(* Logix 5000 Rung export; software revision 16.04 *)

MODULES
   Local : vendor None type None code None
   DNPNET : vendor None type None code None
END_MODULES

TYPE DNPNET_A32in_ClassDeadband_Override :   // List entry for Analog32 Input Class and Deadband Override
STRUCT
   Point_Number : INT;   // Point number to assign class and deadband to.
   Class : INT;   // Class value (1-3)
   Deadband : DINT;   // Deadband for given point number
END_STRUCT
END_TYPE

TYPE DNPNET_CROBmsg_Handler :   // Handles the processing of CROB Messages from Remote Client
STRUCT
   OneShot : BOOL;
   CountPerBlock : INT;   // Number of CROB messages from the Remote Client in in the last 9910 block of multiple blocks.
   CCC : DINT;   // Continuous Crob message Count that may be reset by the User. Otherwise it will cycle from 0 to the DINT type upper limit
   CCBC : DINT;   // Continuous Crob Message Block Count that may be reset by the User. Otherwise it will cycle from 0 to the DINT type upper limit
END_STRUCT
END_TYPE

TYPE DNPNET_Server_List :   // List entry to define an IED unit and its specific communication parameters for a DNP Client port
STRUCT
   Address : INT;
   Data_Link_Confirm_Mode : INT;
   Data_Link_Confirm_Timeout : INT;
   Data_Link_Confirm_Retries : INT;
   Application_Layer_Response_Timeout : INT;
   Server_Mode : INT;   // Bit 0: Enable; Bit 1: Unsol. Msg; Bit 2: Delay Meas; Bit 3: Auto Time Sync; Bit 4: Time Sync Var (0=Var3, 1=Var1)
   IP_Address : DNPNET_WhiteList_IP_address;
   Port : DINT;
   IP_Type : INT;
   Connection_Retry_Interval : INT;
END_STRUCT
END_TYPE

TYPE DNPNETSTATUS :   // This structure encapsulates all the status and scratch variables used by the MVI56E-DNPNET module.
STRUCT
   GenStat : DNPNET_Server_Status;   // General status information
   ErrorList : INT[60];   // List of last 60 DNPNET module errors
   IINServerBits : INT[40];   // IIN Bits received from Servers
   ServerCommErrors : DNPNET_Server_Comm_Error_Element[40];   // Server communication errors list
   CommandErrors : INT[300];   // Command errors list
   Network : DNPNET_Network;
END_STRUCT
END_TYPE

TYPE DNPNET_Command_Error_Request :   // this goes into a 9950 block to request command errors
STRUCT
   Request : BOOL;   // send a 9950 command error request block
   Number_Of_Commands : INT;   // Number of commands to report (1 - 200)
   Start_Index : INT;   // Index in the command list to start
END_STRUCT
END_TYPE

TYPE DNPNETCONTROL :
STRUCT
   Events : DNPNET_EventsHandler;   // Handling the transfer of events from the Events Message Buffer in the Client to the PLC
   EventMessages : DNPNET_EventMessage[15];   // Events Captured by DNP Client are moved to this structure
   CROBmsg_counter : DNPNET_CROBmsg_Handler;   // Number of block 9910 CROB messages from DNP Server
   CROBmsg_data : DNPNET_CROB_Data[40];   // CROB message data copied via block 9910 from DNP Server
   Binary_Event_CalTime : DNPNET_Event_Binary_CalTime;   // For storing block 9958 Binary Input Events with CAL time to be sent by DNP Server
   Analog_Event_CalTime : DNPNET_Event_Analog_CalTime;   // For storing block 9959 Analog Input Events with CAL time to be sent by DNP Server
   Binary_Event_CLXTime : DNPNET_Event_Binary_CLXTime;   // For storing Block 9968 Binary Input Events with CLX Time to be sent by DNP server
   Analog_Event_CLXTime : DNPNET_Event_Analog_CLXTime;   // For storing Block 9969 Binary Input Events with CLX Time to be sent by DNP server
   Get_Module_Time : DNPNET_Module_Time_Get;
   Set_Module_Time : DNPNET_Module_Time_Set;
   CROB_Commands : DNPNET_CROB_Commands;   // 9901 block of CROB Commands
   Aux_Commands : DNPNET_Aux_Command;   // 9904 block for Auxiliary Client commands
   CommandControl : DNPNET_Command_Control;   // 9902 block of commands to enable
   Server_Comm_Errors : DNPNET_Server_Error_Request;   // count and offset of servers to report
   Command_Errors : DNPNET_Command_Error_Request;   // count and offset of commands to report
   ColdBoot : BOOL;   // Cold boot the DNP module via block 9999
   WarmBoot : BOOL;   // Warm boot the DNP module via block 9998
   ChangeDatabaseSize : BOOL;   // Manual bit to change database size
END_STRUCT
END_TYPE

TYPE DNPNET_CROB_Command_Element :   // This is a single CROB command for a CROB command block
STRUCT
   Port_Flag : INT;   // ignored
   Server_Address : INT;   // Address of server to be controlled
   Object : INT;   // Object type 12
   Variation : INT;   // Variation1
   Function : INT;   // Function 3, 5, or 6
   Point_Number_In_Server : INT;   // Point number in the IED to be controlled
   Control_Code : INT;   // Standard DNP control code byte
   Pulse_Count : INT;   // Number of pulses from 0 to 255
   Pulse_On : INT;   // Pulse on time interval
   Pulse_Off : INT;   // Pulse off time interval
END_STRUCT
END_TYPE

TYPE DNPNET_Event_Analog_CalTime :   // Holds binary input events with calendar time block 9959
STRUCT
   Send : BOOL;   // Sends block 9959 Analog_Event messages to DNP Server
   Event_Count : INT;   // Number of events (1 to 20)
   Sequence_Counter : INT;   // Sequence counter for each block transfer, used to synchronize and confirm receipt of the block by the module
   Event : DNPNET_Event_Analog_CalTime_Element[20];   // Analog input events to be transferred to the module
   Event_Count_Rec : INT;   // Number of events (1 - 20) received
   Seq_Count_Rec : INT;   // Sequence counter Received for each block transfer, used to synchronize and confirm receipt of the block by the module
END_STRUCT
END_TYPE

TYPE DNPNET_Event_Binary_CLXTime_Element :   // Block 9968 binary CLXTime event element
STRUCT
   Point_Number : INT;   // Point number in the DNP binary input database
   Class_Override : INT;   // Bits 0 and 1 are used for class override values of 1 to 3
   Value : INT;   // Bit 0 = digital state for point. ALL other bits are ignored
   reserved : INT;
   CLX_Time : LINT;   // 64-bit Time as number of microseconds since Jan 1st, 1970
END_STRUCT
END_TYPE

TYPE DNPNET_DBLin_ClassDeadband_Override :   // List entry for Double Float Input Class and Deadband Override
STRUCT
   Point_Number : INT;   // Point number to assign class and deadband to
   Class : INT;   // Class value (1-3)
   Deadband : REAL;   // Deadband for given point number
END_STRUCT
END_TYPE

TYPE DNPNET_Server_Comm_Error_Element :   // Server communication errors
STRUCT
   Index : INT;   // index in the module's server list
   Server_Address : INT;   // DNP server address for the device
   Bad_CRC : INT;   // number of bad CRCs received from the server
   Buffer_Overflow : INT;   // number of buffer overflow messages received from the server
   Trans_Seq_Num : INT;   // the number of incorrect transport sequence errors
   Confirm_Retry : INT;   // number of data link layer confirm request retries
   Confirm_Fail : INT;   // number of data link layer confirm request failures
   No_App_Resp : INT;   // number of application layer no responses to requests
END_STRUCT
END_TYPE

TYPE DNPNET_WhiteList_IP_address :   // Structure containing the four octets for White List IP addresses
STRUCT
   a : INT;   // a . XXX . XXX . XXX
   b : INT;   // XXX . b . XXX . XXX
   c : INT;   // XXX . XXX . c . XXX
   d : INT;   // XXX . XXX . XXX . d
END_STRUCT
END_TYPE

TYPE DNPNET_Client_Parameters :   // This structure contains configuration parameters for the DNP client
STRUCT
   Internal_ID : INT;   // Client's Identification Number
   Event_Messages_to_PLC : INT;
   Initialize_IED_Input_Database : INT;
   Only_Time_Sync_Servers_If_Synced : INT;
   Use_Binary_Output_status_Data : INT;
   Use_Analog_Output_status_Data : INT;
   Dont_Process_IIN : INT;
   reserved_0 : INT;
END_STRUCT
END_TYPE

TYPE DNPNET_Module_Time_Set :   // Write to Module's System TIme
STRUCT
   Send : BOOL;   // Send block 9971 Time from the PLC to the DNP module
   PLC_Time : DINT[7];   // WallclockTime is copied to this tag before being sent to DNP Module
END_STRUCT
END_TYPE

TYPE DNPNET_Client_Commands :   // List entry for commands to process on the master port
STRUCT
   Port_Flags : INT;   // Bit 2:(0=Disable Cmd, 1=Enable Cmd); Bit 3:(0=Poll, 1=Exception); Bit 4:(0=DNP DB, 1=IED DB). Bits 3/4 apply to BO/AO only.
   Server_Address : INT;   // address of server command is sent to
   Object : INT;   // Object number
   Variation : INT;   // Variation number
   Function : INT;   // Function number
   Point_Number_in_Server : INT;   // starting point for request in server
   Point_Count : INT;   // number of points requested in server
   DNP_DB_Point_Number_in_Client : INT;   // starting point in DNP database for storing response
   IED_DB_Point_Number_in_Client : INT;   // starting point in IED database for storing response
   Poll_Interval : INT;   // how often to send command
END_STRUCT
END_TYPE

TYPE DNPNET_IED_DB_Definitions :   // This structure contains CALCULATED Point Counts/Sizes used by the IED Database. NOT editable by user.
STRUCT
   Binary_Input_Words : INT;   // number of Object 1 words (points * 16)
   Analog16_Inputs : INT;   // number of Object 30 INTs
   Analog32_Inputs : INT;   // number of Object 30 DINTs
   Float_Inputs : INT;   // number of Object 30 REALs
   Counters : INT;   // number of Object 20 DINTs
   Binary_Output_Words : INT;   // number of Object 12 words (points * 16)
   Analog16_Outputs : INT;   // number of Object 41 INTs
   Analog32_Outputs : INT;   // number of Object 41 DINTs
   Float_Outputs : INT;   // number of Object 41 REALs
   Binary_Out_Words_Status_Size : INT;   // number of Object 10 words (points * 16)
   Analog16_Out_Status_Size : INT;   // number of Object 40 INTs
   Analog32_Out_Status_Size : INT;   // number of Object 40 DINTs
   Float_Out_Status_Size : INT;   // number of Object 40 REALs
   reserved_0 : INT;
END_STRUCT
END_TYPE

TYPE DNPNET_IED_Output_Database :
STRUCT
   Binary : INT[100];   // Object 12 binary INTs for Remote Server's database
   Analog16 : INT[100];   // Object 41 analog INTs for Remote Server's database
   Analog32 : DINT[50];   // Object 41 analog DINTs for Remote Server's database
   Float : REAL[50];   // Object 41 analog REALs for Remote Server's database
END_STRUCT
END_TYPE

TYPE DNPNET_Server_DB_Points :   // This structure contains Point Counts used by the DNP Server Database
STRUCT
   Binary_Input_Words : INT;   // number of Object 1 words (points * 16)
   PLC_Binary_Input_Words : INT;   // number of Object 1 words (points * 16) to be shared with PLC
   Analog_Inputs : INT;   // number of Object 30 INTs
   PLC_Analog_Inputs : INT;   // number of Object 30 INTs to be shared with PLC
   Analog32_Inputs : INT;   // number of Object 30 DINTs
   PLC_Analog32_Inputs : INT;   // number of Object 30 DINTs to be shared with PLC
   Float_Inputs : INT;   // number of Object 30 REALs
   PLC_Float_Inputs : INT;   // number of Object 30 REALs to be shared with PLC
   Double_Inputs : INT;   // number of Object 30 double precision floats
   PLC_Double_Inputs : INT;   // number of Object 30 double precision floats to be shared with PLC
   Counters : INT;   // number of Object 20 DINTs
   PLC_Counters : INT;   // number of Object 20 DINTs to be shared with PLC
   Binary_Output_Words : INT;   // number of Object 12 words (points * 16)
   PLC_Binary_Output_Words : INT;   // number of Object 12 words (points * 16) to be shared with PLC
   Analog_Outputs : INT;   // number of Object 41 INTs
   PLC_Analog_Outputs : INT;   // number of Object 41 INTs to be shared with PLC
   Analog32_Outputs : INT;   // number of Object 41 DINTs
   PLC_Analog32_Outputs : INT;   // number of Object 41 DINTs to be shared with PLC
   Float_Output : INT;   // number of Object 41 REALs
   PLC_Float_Outputs : INT;   // number of Object 41 REALs to be shared with PLC
   Double_Outputs : INT;   // number of Object 41 Double precision floats
   PLC_Double_Outputs : INT;   // number of Object 41 Double precision floats to be shared with PLC
   Disable_Points : DNPNET_Disable_DNP;   // Allows for DNP datatypes to be disabled, which removes them from the server database.
END_STRUCT
END_TYPE

TYPE DNPNET_CROB_Data :   // This object encapsulates the data for the DNP CROB (slave)
STRUCT
   Point_Number : INT;   // point number to be controlled
   Control_Code : SINT;   // standard DNP control code byte
   count : SINT;   // number of pulses
   On_Time : DINT;   // on time interval
   Off_Time : DINT;   // off time interval
END_STRUCT
END_TYPE

TYPE DNPNET_EventMessage :   // Event message received by the Client and passed to ladder logic.
STRUCT
   Device_Index : INT;   // Server list index where event came from
   IED_Address : INT;   // IED database index where the data was stored
   DNP_Address : INT;   // DNP database index where the data was stored
   Server_Address : INT;   // Server (IED) address which generated the event
   Point_Number : INT;   // point number of the data that changed in the IED
   Object : INT;   // DNP object number for point
   Variation : INT;   // DNP variation for event
   reserved : INT;
   Time : LINT;   // DNP time of the event
   DINT_Value : DINT;   // INT or DINT value of the data
   REAL_Value : REAL;   // REAL value of the data
END_STRUCT
END_TYPE

TYPE DNPNET_DNP_Input_Database :
STRUCT
   Binary : INT[100];   // Object 1 binary INTs for Server's database
   Analog16 : INT[100];   // Object 30 analog INTs for Server's database
   Analog32 : DINT[50];   // Object 30 analog DINTs for Server's database
   Float : REAL[50];   // Object 30 analog REALs for Server's database
   Double : DNPNET_Double_Type_Data[50];   // Object 30 analog double precision floats for Server's database
   Counter : DINT[50];   // Object 20 counter DINTs for Server's database
END_STRUCT
END_TYPE

TYPE DNPNET_Event_Analog_CLXTime_Element :   // Block 9969 Analog CLXTime event element
STRUCT
   Point_Number : INT;   // Data Point in the DNP analog input database
   Class_Override : INT;   // Bits 0 and 1 are used for class override values of 1 to 3
   Value : DINT;   // input value
   CLX_Time : LINT;   // CLX Time as number of microseconds since Jan 1 1970
END_STRUCT
END_TYPE

TYPE DNPNET_Server_Parameters :   // This structure contains configuration parameters for the DNP server
STRUCT
   Internal_Server_ID : INT;   // DNP address for the module
   Use_WhiteList : INT;   // Parameter specifies if the IP address of host will be validated. 0 = Any List, 1 = Use Whitelist
   Binary_Input_Class : INT;   // Parameter specifies the default class to be utilized for all the Binary Input points
   Analog16_Input_Class : INT;   // Parameter specifies the default class to be utilized for all 16-bit Analog Input points
   Analog32_Input_Class : INT;   // Parameter specifies the default class to be utilized for all 32-bit Analog Input points
   Float_Class : INT;   // Parameter specifies the default class to be utilized for all the Float Input points
   Double_Class : INT;   // Parameter specifies the default class to be utilized for all the Double Input points
   Analog16_Input_Deadband : INT;   // Parameter specifies the default deadband value assigned to all points not defined in the override list
   Analog32_Input_Deadband : DINT;   // Parameter specifies the default deadband value assigned to all points not defined in the override list
   Float_Deadband : REAL;   // Parameter specifies the default deadband value assigned to all points not defined in the override list
   Double_Deadband : REAL;   // Parameter specifies the default deadband value assigned to all points not defined in the override list
   SelectOperate_Arm_Time : INT;   // Time period after select command is received in which operate command will be performed (in milliseconds)
   Write_Time_Interval : INT;   // Time interval to set the need time IIN bit. 0 = Never (in minutes)
   Data_Link_Confirm_Mode : INT;   // Request acknowledgement from Client station. Default = 0 (recommended)
   Data_Link_Confirm_Tout : INT;   // Time period to wait for Client Data Link confirmation of last frame sent. Default = 1000 (recommended)
   Data_Link_Max_Retry : INT;   // Maximum number of retries at the Data Link level to obtain a confirmation. Default = 2 (recommended)
   App_Layer_Confirm_Tout : INT;   // Event data contained in the last response may be sent again if not confirmed (in milliseconds)
   Unsolicited_Response : INT;   // 0 = Server will not send unsolicited responses; 1 = Server will send unsolicited responses
   Class_1_Unsol_Resp_Min : INT;   // Minimum number of events in Class 1 required before an unsolicited response will be generated.
   Class_2_Unsol_Resp_Min : INT;   // Minimum number of events in Class 2 required before an unsolicited response will be generated.
   Class_3_Unsol_Resp_Min : INT;   // Minimum number of events in Class 3 required before an unsolicited response will be generated.
   Unsol_Resp_Delay : INT;   // Maximum number of milliseconds to wait after an event occurs before sending an unsolicited response message
   UResp_Client_Address : INT;   // DNP destination address where unsolicited response messages are sent
   AnalogIinput_Events_with_time : INT;   // Parameter that sets if the Analog Input event will include date and time; 0 = without DateTime; 1 = With DateTime
   Events_Require_Time_Sync : INT;   // Parameter is used to determine if events will be generated if time is not synched. 0 = events generated; 1 = no events generated
   Initialize_DNP_Output_Database : INT;   // Parameter determines if the module will request data from the processor to initialize DNP database output data
   PassThrough_CROB : INT;   // Parameter determines if module will pass all received CROB messages received through processor. (see User Manual for more info)
   Use_TripClose_Single_Point : INT;   // Parameter determines if data associated with CROB commands operate on single or dual point. (see User Manual for more info)
   Unsol_Retry_Limit : INT;   // Configurable unsolicited retry limit. Range = 7 to 32768
   Use_SOE_card : BOOL;   // Using Allen Bradly 1756-SOE Sequence Of Events Module. 0=No, 1=Yes
   Use_Data_from_Client_connection : BOOL;   // Set this option to to allow data from MVI client connection to be shared with MVI server database. 0 = disable; 1 = enable
   Use_Double_Floats : BOOL;   // Set this option to to use the DNP Double Float (64bit) database. 0 = disable; 1 = enable
   Block_Timeout_MS : INT;   // Backplane block heartbeat. Range = 11 to 5000, default = 1500 (in milliseconds)
   Server_Timeout : INT;   // Configurable TCP server connection timeout parameter. Range = 5 to 32767 (in seconds)
   Port : INT;   // Configurable Server Port parameter. Range = 0-32767
END_STRUCT
END_TYPE

TYPE DNPNET_Event_Binary_CLXTime :   // Block 9968
STRUCT
   Send : BOOL;   // Send block 9968 Binary event with CLX time to DNP Server
   Event_Count : INT;   // Number of events in the block (1 to 30)
   Sequence_Counter : INT;   // Used to set and synchronize and confirm receipt of the block by the module.
   Event : DNPNET_Event_Binary_CLXTime_Element[30];   // Events
   Event_Count_Rec : INT;   // Number of events (1 - 30) received
   Seq_Count_Rec : INT;   // Used to synchronize and confirm receipt of the block by the module.
END_STRUCT
END_TYPE

TYPE DNPNET_FLTin_ClassDeadband_Override :   // List entry for Float Input Class and Deadband Override
STRUCT
   Point_Number : INT;   // Point number to assign class and deadband to.
   Class : INT;   // Class value (1-3)
   Deadband : REAL;   // Deadband for given point number
END_STRUCT
END_TYPE

TYPE DNPNET_Server_Status :   // This object contains the status information for the DNP Server
STRUCT
   Cur_Port : INT;   // Current DNP Slave port
   Last_Err : INT;   // Last DNP slave error code
   Msg_Me : INT;   // Total message frames for slave
   Msg_Sent : INT;   // Total message frames sent
   Msg_Rec : INT;   // Total message frames received
   Err_Sync : INT;   // Total number of synchronization errors
   Err_Overrun : INT;   // Total number of over runs errors
   Err_Length : INT;   // Total number of length errors
   Err_CRC : INT;   // Total number of CRC errors
   Err_Overflow : INT;   // Total number of overflow errors
   Err_Seq : INT;   // Total number of sequence errors
   Err_Address : INT;   // Total multi-frame request fragment errors
   Err_Func : INT;   // Total number of bad function errors
   Err_Obj : INT;   // Total number of object unknown errors
   Err_Range : INT;   // Total number of range errors
   Err_MOverflow : INT;   // Total number of app msg overflow errors
   Err_Frame : INT;   // Total number of multi-frame errors
   Blk_Err : INT;   // Total number of blocks in error
   Blk_Good : DINT;   // Total number of blocks transferred successfully
   Blk_RErr : INT;   // Total number of read block errors
   Blk_WErr : INT;   // Total number of write block errors
   Blk_NErr : INT;   // Total number of block number errors
   Blk_ECntr : INT;   // Number of sequential block errors
   Blk_EFlag : INT;   // Block error flag
   Cfg_Type : INT;   // 0=Single Slave, 1-Dual-Slave, 2=Slave/Master
   Product : SINT[4];   // Product name
   Rev : SINT[4];   // Revision
   Op_Sys : SINT[4];   // Operating system revision
   Run : SINT[4];   // Run number
   Slave_Count : INT;   // Number of slaves configured
   Cmd_Count : INT;   // Number of commands configured
   Mem_Blk : INT;   // Number of memory blocks allocated
   Mem_Frame : INT;   // Number of frame blocks allocated
   Mem_DLRec : INT;   // Number of receive DL blocks allocated
   Mem_DLTx : INT;   // Number of transmit DL blocks allocated
   Mem_AppRec : INT;   // Number of receive app blocks allocated
   Mem_AppTx : INT;   // Number of transmit app blocks allocated
   Mem_DevErr : INT;   // Number of device mem alloc errors
   Mem_PhyErr : INT;   // Number of physical layer mem alloc errors
   Mem_DLRErr : INT;   // Number of data-link layer receive mem alloc errors
   Mem_DLTErr : INT;   // Number of data-link layer transmit mem alloc errors
   Mem_AppRErr : INT;   // Number of app layer receive mem alloc errors
   Mem_AppTErr : INT;   // Number of app layer transmit mem alloc errors
   Mstr_Sync : INT;   // Number of master port synchronization errors
   Mstr_Length : INT;   // Number of master port length errors
   Mstr_CRC : INT;   // Number of master port CRC errors
   P1_TX_State : INT;   // State of Port 1 transmit state machine
   Scan_Count : DINT;   // Program scan counter
   Mem_Free : DINT;   // Free memory for module
   BI_Events : INT;   // Total number of BI events
   BI_Buffer : INT;   // Total number of BI events in buffer
   AI_Events : INT;   // Total number of AI events
   A16I_Buffer : INT;   // Total number of AI events in buffer
   A32I_Events : INT;   // Analog 32-bit INT input events total
   A32I_Buffer : INT;   // Analog 32-bit INT input events in server queue
   FLTI_Events : INT;   // Count of floating-point events
   FLTI_Buffer : INT;   // Analog float input events in queue
   DBLI_Events : INT;   // Count of double floating-point events
   DBLI_Buffer : INT;   // Analog double float input events in queue
   Events_In_Client : INT;   // Total number of events in message queue for processor
   Events_In_Client_OF : INT;   // Event message queue overflow flag (0=no, 1=yes)
   Slave_IIN_Bits : INT;   // Local slave IIN bits being reported to controlling station
   reserved : INT;
END_STRUCT
END_TYPE

TYPE DNPNETCONFIG :   // This structure contains the different members of the config structure
STRUCT
   DNP_Module_Name : SINT[40];   // String of ASCII characters that gives the module a unique name. Terminate the string with a byte = 0.
   DNP3_Server : DNPNET_Server_Parameters;   // DNPNET Server Configuration
   DNP3_WhiteList : DNPNET_WhiteList_IP_address[10];   // IP addresses of the Clients that the Server will respond to.
   DNP3_Client : DNPNET_Client_Parameters;   // DNPNET Client Configuration
   DNP_Server_Override : DNPNET_Override;   // For assigning Class and Deadband overrides to individual point types.
   DNP_Server_List : DNPNET_Server_List[5];   // List of Servers the Client connects to
   DNP_Client_Commands : DNPNET_Client_Commands[5];   // List of commands the Client send to Servers
   IP_Settings : DNPNET_Module_IP_Addressing;   // Assigns the IP address configuration of the MVI56E-DNPNET
END_STRUCT
END_TYPE

TYPE DNPNET_Event_Binary_CalTime :   // Holds binary input events with calendar time block 9958.
STRUCT
   Send : BOOL;   // Sends block 9958 Binary_Event messages to DNP Server
   Event_Count : INT;   // Number of events (1 - 24)
   Sequence_Counter : INT;   // Sequence counter for each block transfer, used to synchronize and confirm receipt of the block by the module
   Event : DNPNET_Event_Binary_CalTime_Element[24];   // Binary input events to be transferred to the module
   Event_Count_Rec : INT;   // Number of events (1 - 24) received
   Seq_Count_Rec : INT;   // Sequence counter Received for each block transfer, used to synchronize and confirm receipt of the block by the module
END_STRUCT
END_TYPE

TYPE DNPNET_DNP_Output_Database :
STRUCT
   Binary : INT[100];   // Object 12 binary INTs from Server's database
   Analog16 : INT[100];   // Object 41 analog INTS from Server's database
   Analog32 : DINT[50];   // Object 41 analog DINTs from Server's database
   Float : REAL[50];   // Object 41 analog REALs from Server's database
   Double : DNPNET_Double_Type_Data[50];   // Object 41 analog double precision floats from Server's database
END_STRUCT
END_TYPE

TYPE DNPNET_Double_Type_Data :   // This object encapsulates an Input and Output 8 BYTE data array.
STRUCT
   Data : SINT[8];   // 8 byte input and output array
END_STRUCT
END_TYPE

TYPE DNPNET_Disable_DNP :   // This structure allows for some DNP datatypes to be disabled, which removes them from the server database.
STRUCT
   Disable_DNP_BI : BOOL;   // Disables DNP Binary Inputs.
   Disable_DNP_AI_16 : BOOL;   // Disables DNP Analog INT Inputs.
   Disable_DNP_AI_32 : BOOL;   // Disables DNP Analog DINT Inputs.
   Disable_DNP_FI : BOOL;   // Disables DNP Float Inputs.
   Disable_DNP_Counters : BOOL;   // Disables DNP Counters.
   Disable_DNP_BO : BOOL;   // Disables DNP Binary Outputs.
   Disable_DNP_AO_16 : BOOL;   // Disables DNP Analog INT Outputs.
   Disable_DNP_AO_32 : BOOL;   // Disables DNP Analog DINT Outputs.
   Disable_DNP_FO : BOOL;   // Disables DNP Float Outputs.
END_STRUCT
END_TYPE

TYPE DNPNET_IED_Input_Database :
STRUCT
   Binary : INT[100];   // Object 1 binary INTs from Client's database
   Analog16 : INT[100];   // Object 30 analog INTs from Client's database
   Analog32 : DINT[50];   // Object 30 analog DINTs from Client's database
   Float : REAL[50];   // Object 30 analog REALs from Client's database
   Counter : DINT[50];   // Object 20 counter DINTs from Client's database
   Binary_Out_Status : INT[100];   // Object 10 INTs. Output Status from Client's database
   Analog16_Out_Status : INT[100];   // Object 10 INTs. Output Status from Client's database
   Analog32_Out_Status : DINT[50];   // Object 40 analog DINTs. Output Status from Client's database
   Float_Out_Status : REAL[50];   // Object 40 analog REALs. Output Status from Client's database
END_STRUCT
END_TYPE

TYPE DNPNET_Module_Time_Get :   // Read Module's System TIme
STRUCT
   Request : BOOL;   // Request block 9970 time from the DNP module
   Set_PLC_Time : BOOL;   // Allow time from the Module to set the PLC clock
   Clock : DNPNET_Clock;   // For storing block 9970 Time from DNP Server
END_STRUCT
END_TYPE

TYPE DNPNET_Event_Binary_CalTime_Element :   // Events with calendar time to be packed into block 9958
STRUCT
   Point_Number : INT;   // Data point in the DNP binary database represented by event
   Class_Override : INT;   // Class Override Value (1 through 3)
   Value : INT;   // Point Value
   Year : INT;   // Year
   Month : INT;   // Month
   Day : INT;   // Day
   Hour : INT;   // Hour
   Minute : INT;   // Minute
   Seconds : INT;   // Seconds
   Milliseconds : INT;   // Milliseconds
END_STRUCT
END_TYPE

TYPE DNPNET_EventsHandler :   // Handles the transferring of Event Messages from the Client to the PLC.
STRUCT
   OneShot : BOOL;
   CountPerBlock : INT;   // Number of events per block 9903 from DNP Client to EventMsgs structure
   BufferOverflow : INT;   // Indicates if Client Event Messages buffer has overflowed when Client received Event Messages from the remote Server
   Queued : INT;   // Number of Events remaining in DNP Client's Event Message buffer at the time of PLC's reading the current 9903 Block
   CountTotal : INT;   // Number of Event Messages retrieved from remote Server and currently present in Events Message Buffer
   BlockTransferCount : INT;   // Number of times that the quantity of Event Messages in the Buffer had to be read by the PLC through the backplane
   BTCountTotal : INT;   // Block Transfer Count Total
   CEC : DINT;   // Continuous Events Count. Keeps counting Events until user reset or count limit recycles.
   CBC : DINT;   // Continuous Block Count. Keeps counting 9903 blocks until user reset or count limit recycles.
END_STRUCT
END_TYPE

TYPE DNPNET_Command_Control :   // Controlling DNPNET Commands
STRUCT
   Send : BOOL;   // Send a command control block 9902
   NumberofCommands : INT;   // The number of commands to Enable
   ClientCommands : INT[240];   // The numbers of the commands in the Client Command List to enable
END_STRUCT
END_TYPE

TYPE DNPNET_Server_Error_Request :   // Request server communication errors via this 9949 block
STRUCT
   Request : BOOL;   // send a 9949 Server communication error request block
   Number_of_Servers : INT;   // number of servers to report in the response message
   Server_Start_Index : INT;   // index in slave list to start
END_STRUCT
END_TYPE

TYPE DNPNET_Network :   // Server TCP/ UDP Network Status
STRUCT
   TCP_Parsing : INT;   // Indication of TCP Parsing: -1 = Offline, 0 = No, 1 = Yes
   Multi_Frag : INT;   // Multi-Fragment Message Indicator: 0 = No, 1 = Yes
   Transport_Frag : INT;   // Transport Fragmented Message Indicator
   Confirm_Pend : INT;   // Confirmation Pending Indicator: 0 = No, 1 = Yes
   TCP_Rx_Count : INT;   // TCP Message Received Count
   TCP_Tx_Count : INT;   // TCP Message Transmitted Count
   Tx_State : INT;   // Module Transmit State
   TCP_State : INT;   // TCP Communication State: 0 = Not Communicating using TCP, 1 = Communicating using TCP, 2 = Received Multi-Message Packet
   Busy_Flag : INT;   // Communication Busy Indicator: 0 = Not Busy, 1 = TCP Busy, 2 = UDP Busy
   App_Frame : INT;   // Application Frame Fragmented Message Indicator: 0 = No, 1 = Yes
   Tx_Frame : INT;   // Transmit Frame State
   TCP_PacketLength : INT;   // Packet Length of TCP Message
   UDP_Parsing : INT;   // Indication of UDP Parsing: 0 = No, 1 = Yes
   UDP_Rx_Count : INT;   // UDP Message Received Count
   UDP_Tx_Count : INT;   // UDP Message Transmitted Count
   UDP_State : INT;   // UDP Communication State: 0 = Not Communicating using UDP, 1 = Communicating using UCP
   UDP_PacketLength : INT;   // Packet Length of UDP Message
END_STRUCT
END_TYPE

TYPE DNPNET_A16in_ClassDeadband_Override :   // List entry for Analog Input Class and Deadband Override
STRUCT
   Point_Number : INT;   // Point number to assign class and deadband to.
   Class : INT;   // Class Value (1-3)
   Deadband : INT;   // Deadband for given point number
   reserved : INT;
END_STRUCT
END_TYPE

TYPE DNPNET_BinIn_Class_Override :   // List entry for Binary Input Class Override
STRUCT
   Point_Number : INT;   // Point number to assign a Class to.
   Class : INT;   // Class value (1-3)
END_STRUCT
END_TYPE

TYPE DNPNETUTIL :
STRUCT
   LastRead : INT;   // Index of last read block
   LastWrite : INT;   // Index of last write block
   BlockIndex : DINT;   // Computed block offset for data table
   ReadData : INT[50500];   // Buffer File for data Read from Module
   WriteData : INT[30000];   // Buffer File for data Written to Module
   OffsetCounter : DINT;   // For calculating buffer copy offset
   CopyLength : INT;   // For calculating buffer copy length
   LastService : INT;   // For keeping track of last special outgoing block serviced
   Mutex : INT;   // Only one special block gets serviced every other scan
   OddScan : INT;   // Keep track of every other scan
   FirstRun : INT;   // Ensures database counts are correct every time the PLC restarts
   DNP_List_Entry_Counts : DNPNET_List_Entry_Counts;   // lengths of the following seven lists
   IED_Database : DNPNET_IED_DB_Definitions;   // Configure the Client database sizes
   DNP_Server_Database : DNPNET_Server_DB_Points;   // Configured Server database sizes
END_STRUCT
END_TYPE

TYPE DNPNET_Module_IP_Addressing :   // Reads and Writes the IP settings
STRUCT
   Read : BOOL;   // Get Ethernet configuration from the module.
   Write : BOOL;   // Set Ethernet configuration for the module
   IP : INT[4];   // Internet Protocol Octets
   Netmask : INT[4];   // Netmask Octets
   Gateway : INT[4];   // Gateway Octets
   Speed : INT;   // 0=Auto, 10=10Mb, 100=100Mb. Other values default to Auto.
   Duplex : INT;   // 0=Half, 1=Full. Other values default to Auto.
END_STRUCT
END_TYPE

TYPE DNPNET_CROB_Commands :   // A block of CROB commands to send to the DNP module
STRUCT
   Send : BOOL;   // send a 9901 CROB Command block to the DNP module
   Command_Count : INT;   // Number of CROB commands in this block
   CROB_Commands : DNPNET_CROB_Command_Element[24];   // CROB Commands
END_STRUCT
END_TYPE

TYPE DNPNET_Override :
STRUCT
   Binary_Inputs : DNPNET_BinIn_Class_Override[10];   // for assigning classes Overrides to individual points
   Analog16_Inputs : DNPNET_A16in_ClassDeadband_Override[10];   // for assigning class and/or deadband Overrides to individual points
   Analog32_Inputs : DNPNET_A32in_ClassDeadband_Override[10];   // for assigning class and/or deadband Overrides to individual points
   Float_Inputs : DNPNET_FLTin_ClassDeadband_Override[10];   // for assigning class and/or deadband Overrides to individual points
   Double_Inputs : DNPNET_DBLin_ClassDeadband_Override[10];   // for assigning class and/or deadband Overrides to individual points
END_STRUCT
END_TYPE

TYPE DNPNETMODULEDEF :
STRUCT
   CONFIG : DNPNETCONFIG;   // DNPNET module configuration parameters for blocks 9000 - 9099
   DATA : DNPNETDATA;   // Server and Client Databases
   STATUS : DNPNETSTATUS;   // Status Tags for various functionalities
   CONTROL : DNPNETCONTROL;   // Tags for Controlling module's functionality
   UTIL : DNPNETUTIL;   // Tags that perform background tasks
END_STRUCT
END_TYPE

TYPE DNPNET_List_Entry_Counts :   // Contains the number of entries for each variable length DNP configuration list
STRUCT
   BI_Class_Overrides : INT;
   AI_ClassDeadband_Overrides : INT;
   A32I_ClassDeadband_Overrides : INT;
   FLTI_ClassDeadband_Overrides : INT;
   DBLI_ClassDeadband_Overrides : INT;
   Server_List_Entries : INT;
   Client_Commands : INT;
   reserved_0 : INT;
END_STRUCT
END_TYPE

TYPE DNPNETDATA :
STRUCT
   DNP_Outputs : DNPNET_DNP_Output_Database;   // Module's Server Database. Remote Clients Write into this DB.
   IED_Inputs : DNPNET_IED_Input_Database;   // Module's Client Database. The Client writes data into this DB that it Reads from remote Servers.
   DNP_Inputs : DNPNET_DNP_Input_Database;   // Module's Server Database. Remote Clients Read from this DB.
   IED_Outputs : DNPNET_IED_Output_Database;   // Module's Client Database. The Client reads data from this DB and Writes it to remote Servers.
END_STRUCT
END_TYPE

TYPE DNPNET_Clock :   // Stores the date and time information for clock synchronization
STRUCT
   Year : DINT;   // Year returned from GSV to processor
   Month : DINT;   // Month returned from GSV to processor
   Day : DINT;   // Day returned from GSV to processor
   Hours : DINT;   // Hours returned from GSV to processor
   Minutes : DINT;   // Minutes returned from GSV to processor
   Seconds : DINT;   // Seconds returned from GSV to processor
   MicroSeconds : DINT;   // MicroSeconds returned from GSV to processor
   Synchronized : INT;
END_STRUCT
END_TYPE

TYPE DNPNET_Aux_Command :   // Block of commands to send to the DNP Client to operate on time
STRUCT
   Send : BOOL;   // send a 9904 command block to the DNP module
   Command_Count : INT;   // number of commands in this block
   Commands : DNPNET_Command_Element[24];   // commands to send to the DNP Client to operate on time
END_STRUCT
END_TYPE

TYPE DNPNET_Command_Element :   // This is a single Command for a Command Block
STRUCT
   Port_Flag : INT;   // Described in manual
   Server_Address : INT;   // address of server command is sent to
   Object : INT;   // Object number
   Variation : INT;   // Variation number
   Function : INT;   // Function number
   Point_Number_In_Server : INT;   // starting point in server
   Point_Count : INT;   // number of points in server
   DNP_Point_Number_In_Client : INT;   // starting point number in DNP database to store data
   IED_Point_Number_In_Client : INT;   // starting point number in IED database to store data
   reserved : INT;
END_STRUCT
END_TYPE

TYPE DNPNET_Event_Analog_CalTime_Element :   // Events with calendar time to be packed into block 9959
STRUCT
   Point_Number : INT;   // Data point in the DNP analog input database
   Class_Override : INT;   // Class Override Value (1 through 3)
   Value : DINT;   // Point value
   Year : INT;   // Year
   Month : INT;   // Month
   Day : INT;   // Day
   Hour : INT;   // Hour
   Minute : INT;   // Minute
   Seconds : INT;   // Seconds
   Milliseconds : INT;   // Miliseconds
   reserved : INT;
END_STRUCT
END_TYPE

TYPE DNPNET_Event_Analog_CLXTime :   // Block 9969
STRUCT
   Send : BOOL;   // Send block 9969 Analog Event with CLX time to DNP Server
   Event_Count : INT;   // Number of events in the block (1 to 30)
   Sequence_Counter : INT;   // Used to set and synchronize and confirm receipt of the block by the module.
   Event : DNPNET_Event_Analog_CLXTime_Element[30];   // Events
   Event_Count_Rec : INT;   // Number of events (1 - 30) received
   Seq_Count_Rec : INT;   // Used to synchronize and confirm receipt of the block by the module.
END_STRUCT
END_TYPE

ADD_ON_INSTRUCTION AOI56EDNPNET   (* revision 2.6, vendor ProSoft Technology Inc., ExecutePrescan *)
// Add-On MVI56-DNPNET module
// Revision note:
// v2.06: Updated descipritions for DNPNET.CONFIG.DNP_Client_Commands.Port_Flags and DNPNET.CONFIG.DNP3_Server.Write_Time_Interval.
// Help:
// v1.0 - Initial Implementation
// v1.1 - Updated the calculations for Status type points sizes. Update for less setting DB sizes in UDTs only.
// v1.2 - 1)changed AOI for block ID 9968 and block ID 9969 to function correctly 2)added block ID -2 to AOI
// v1.3 - Added DNPNET.CONFIG.DNP3_Server.Unsol_Retry_Limit Controller Tag, Warm/Cold Boot Condition change
// v1.4 -  Added DNPNET.CONFIG.DNP3_Server.Use_Double_Floats, Use_Data_from_Client_Connection and DNP.CONTROL.ChangeDatabaseSize tag
// v1.5 -  Added  DNPNET.STATUS.TcpUdpInfo, Deleted EQU statement and MOV statement on last line on Rung 1 to sent -2 back to firmware
// v1.6 - Changed the default DNPNET.CONFIG.DNP_Server_Override.Analog16_Inputs[5].Point_Number from 0 to 9999
// v1.7 -  Changed the COPY statement destination on TCP Udp Info from DNPNET.STATUS.TcpUdpInfo to  DNPNET.STATUS.TcpUdpInfo.tcp_parsing
// 1.15 - Match firmware version 1.15
// 1.16 - Updated Nework TCP/UDP Descriptions
// 1.17 - Minor update to TCP State Description to include TCP State = 2
// 1.18 - Changed default IP addresses used for Whitelist and ServerList to 0.0.0.0
// 1.19 - Added Server_Timeout parameter to DNPNET.CONFIG.DNP3_Server controller tags
// 1.20 - Changed the DNPNET.CONFIG.DNP3_Server.Server_Timeout default value from 5 to 6
// 2.00 - Added parameter definitions, Increased to v2.0
// 2.01 - Changed Command Enable UDTs/Tags
// 2.02 - Added logic to unlatch send bit and receive event and sequence count for Binary and Analog CAL events, Fixed misspellings.
// 2.03 - Changed Binary_Event_CalTime and Analog_Event_CalTime COPY logic to output tags.
// 2.04 - Renamed DNP3_Server.reserved_0 to DNP3_Server.Port. Added support for custom DNP3 Server Port (0-65535).
// 2.05 - Added logic to disable DNP server datatypes in the database. Updated descriptions for DNP3_Server.Port and DNPNET_Server_List. Updated default value for DNP3_Server.Port to 20000. Added Speed and Duplex fields to DNPNET_Module_IP_Addressing. Updated Source Length to 28 bytes in WriteEthernetMSG.
// 2.06 - Updated descipritions for DNPNET.CONFIG.DNP_Client_Commands.Port_Flags and DNPNET.CONFIG.DNP3_Server.Write_Time_Interval.
VAR_INPUT
   EnableIn1 : BOOL;   // Enable Input - System Defined Parameter
END_VAR
VAR_OUTPUT
   EnableOut1 : BOOL;   // Enable Output - System Defined Parameter
END_VAR
VAR_IN_OUT
   DNPNET : DNPNETMODULEDEF; {required}
   Connection_Input : INT[250]; {required}   // Input parameters.
   Connection_Output : INT[248]; {required}   // Output parameters.
   ReadEthernetMSG : MESSAGE; {required}   // Reads IP Address from the Module
   WriteEthernetMSG : MESSAGE; {required}   // Writes IP Address to the Module
END_VAR
VAR
   MJFAULTS : DINT[12];
   Block_ID_Capture : DINT;
END_VAR

ROUTINE Logic   (* ladder *)
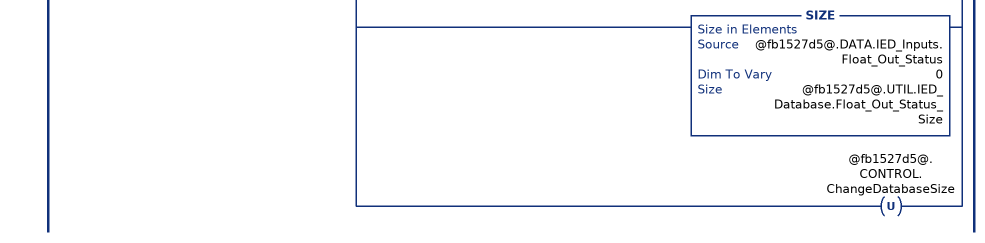
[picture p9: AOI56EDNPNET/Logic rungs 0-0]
   // This rung should only execute once per PLC restart, to ensure that all database size tags are properly populated with values according to database sizes.
   0: [EQU(@fb1527d5@.UTIL.FirstRun,1) ,XIC(@fb1527d5@.CONTROL.ChangeDatabaseSize) ][MOV(0,@fb1527d5@.UTIL.FirstRun) ,[XIO(@fb1527d5@.UTIL.DNP_Server_Database.Disable_Points.Disable_DNP_BI) SIZE(@fb1527d5@.DATA.DNP_Inputs.Binary[0],0,@fb1527d5@.UTIL.DNP_Server_Database.PLC_Binary_Input_Words) ,XIC(@fb1527d5@.UTIL.DNP_Server_Database.Disable_Points.Disable_DNP_BI) MOV(0,@fb1527d5@.UTIL.DNP_Server_Database.PLC_Binary_Input_Words) ,XIO(@fb1527d5@.CONFIG.DNP3_Server.Use_SOE_card) XIO(@fb1527d5@.CONFIG.DNP3_Server.Use_Data_from_Client_connection) MOV(@fb1527d5@.UTIL.DNP_Server_Database.PLC_Binary_Input_Words,@fb1527d5@.UTIL.DNP_Server_Database.Binary_Input_Words) ] ,LES(@fb1527d5@.UTIL.DNP_Server_Database.Binary_Input_Words,@fb1527d5@.UTIL.DNP_Server_Database.PLC_Binary_Input_Words) COP(@fb1527d5@.UTIL.DNP_Server_Database.PLC_Binary_Input_Words,@fb1527d5@.UTIL.DNP_Server_Database.Binary_Input_Words,1) ,[XIO(@fb1527d5@.UTIL.DNP_Server_Database.Disable_Points.Disable_DNP_AI_16) SIZE(@fb1527d5@.DATA.DNP_Inputs.Analog16[0],0,@fb1527d5@.UTIL.DNP_Server_Database.PLC_Analog_Inputs) ,XIC(@fb1527d5@.UTIL.DNP_Server_Database.Disable_Points.Disable_DNP_AI_16) MOV(0,@fb1527d5@.UTIL.DNP_Server_Database.PLC_Analog_Inputs) ,XIO(@fb1527d5@.CONFIG.DNP3_Server.Use_Data_from_Client_connection) MOV(@fb1527d5@.UTIL.DNP_Server_Database.PLC_Analog_Inputs,@fb1527d5@.UTIL.DNP_Server_Database.Analog_Inputs) ] ,LES(@fb1527d5@.UTIL.DNP_Server_Database.Analog_Inputs,@fb1527d5@.UTIL.DNP_Server_Database.PLC_Analog_Inputs) COP(@fb1527d5@.UTIL.DNP_Server_Database.PLC_Analog_Inputs,@fb1527d5@.UTIL.DNP_Server_Database.Analog_Inputs,1) ,[XIO(@fb1527d5@.UTIL.DNP_Server_Database.Disable_Points.Disable_DNP_AI_32) SIZE(@fb1527d5@.DATA.DNP_Inputs.Analog32[0],0,@fb1527d5@.UTIL.DNP_Server_Database.PLC_Analog32_Inputs) ,XIC(@fb1527d5@.UTIL.DNP_Server_Database.Disable_Points.Disable_DNP_AI_32) MOV(0,@fb1527d5@.UTIL.DNP_Server_Database.PLC_Analog32_Inputs) ,XIO(@fb1527d5@.CONFIG.DNP3_Server.Use_Data_from_Client_connection) MOV(@fb1527d5@.UTIL.DNP_Server_Database.PLC_Analog32_Inputs,@fb1527d5@.UTIL.DNP_Server_Database.Analog32_Inputs) ] ,LES(@fb1527d5@.UTIL.DNP_Server_Database.Analog32_Inputs,@fb1527d5@.UTIL.DNP_Server_Database.PLC_Analog32_Inputs) COP(@fb1527d5@.UTIL.DNP_Server_Database.PLC_Analog32_Inputs,@fb1527d5@.UTIL.DNP_Server_Database.Analog32_Inputs,1) ,[XIO(@fb1527d5@.UTIL.DNP_Server_Database.Disable_Points.Disable_DNP_FI) SIZE(@fb1527d5@.DATA.DNP_Inputs.Float[0],0,@fb1527d5@.UTIL.DNP_Server_Database.PLC_Float_Inputs) ,XIC(@fb1527d5@.UTIL.DNP_Server_Database.Disable_Points.Disable_DNP_FI) MOV(0,@fb1527d5@.UTIL.DNP_Server_Database.PLC_Float_Inputs) ,XIO(@fb1527d5@.CONFIG.DNP3_Server.Use_Data_from_Client_connection) MOV(@fb1527d5@.UTIL.DNP_Server_Database.PLC_Float_Inputs,@fb1527d5@.UTIL.DNP_Server_Database.Float_Inputs) ] ,LES(@fb1527d5@.UTIL.DNP_Server_Database.Float_Inputs,@fb1527d5@.UTIL.DNP_Server_Database.PLC_Float_Inputs) COP(@fb1527d5@.UTIL.DNP_Server_Database.PLC_Float_Inputs,@fb1527d5@.UTIL.DNP_Server_Database.Float_Inputs,1) ,XIO(@fb1527d5@.CONFIG.DNP3_Server.Use_Double_Floats) [MOV(0,@fb1527d5@.UTIL.DNP_Server_Database.Double_Inputs) ,MOV(0,@fb1527d5@.UTIL.DNP_Server_Database.PLC_Double_Inputs) ] ,[XIC(@fb1527d5@.CONFIG.DNP3_Server.Use_Double_Floats) SIZE(@fb1527d5@.DATA.DNP_Inputs.Double[0],0,@fb1527d5@.UTIL.DNP_Server_Database.PLC_Double_Inputs) ,XIC(@fb1527d5@.CONFIG.DNP3_Server.Use_Double_Floats) XIO(@fb1527d5@.CONFIG.DNP3_Server.Use_Data_from_Client_connection) MOV(@fb1527d5@.UTIL.DNP_Server_Database.PLC_Double_Inputs,@fb1527d5@.UTIL.DNP_Server_Database.Double_Inputs) ] ,LES(@fb1527d5@.UTIL.DNP_Server_Database.Double_Inputs,@fb1527d5@.UTIL.DNP_Server_Database.PLC_Double_Inputs) COP(@fb1527d5@.UTIL.DNP_Server_Database.PLC_Double_Inputs,@fb1527d5@.UTIL.DNP_Server_Database.Double_Inputs,1) ,[XIO(@fb1527d5@.UTIL.DNP_Server_Database.Disable_Points.Disable_DNP_Counters) SIZE(@fb1527d5@.DATA.DNP_Inputs.Counter[0],0,@fb1527d5@.UTIL.DNP_Server_Database.PLC_Counters) ,XIC(@fb1527d5@.UTIL.DNP_Server_Database.Disable_Points.Disable_DNP_Counters) MOV(0,@fb1527d5@.UTIL.DNP_Server_Database.PLC_Counters) ,XIO(@fb1527d5@.CONFIG.DNP3_Server.Use_Data_from_Client_connection) MOV(@fb1527d5@.UTIL.DNP_Server_Database.PLC_Counters,@fb1527d5@.UTIL.DNP_Server_Database.Counters) ] ,LES(@fb1527d5@.UTIL.DNP_Server_Database.Counters,@fb1527d5@.UTIL.DNP_Server_Database.PLC_Counters) COP(@fb1527d5@.UTIL.DNP_Server_Database.PLC_Counters,@fb1527d5@.UTIL.DNP_Server_Database.Counters,1) ,[XIO(@fb1527d5@.UTIL.DNP_Server_Database.Disable_Points.Disable_DNP_BO) SIZE(@fb1527d5@.DATA.DNP_Outputs.Binary[0],0,@fb1527d5@.UTIL.DNP_Server_Database.PLC_Binary_Output_Words) ,XIC(@fb1527d5@.UTIL.DNP_Server_Database.Disable_Points.Disable_DNP_BO) MOV(0,@fb1527d5@.UTIL.DNP_Server_Database.PLC_Binary_Output_Words) ,XIO(@fb1527d5@.CONFIG.DNP3_Server.Use_Data_from_Client_connection) MOV(@fb1527d5@.UTIL.DNP_Server_Database.PLC_Binary_Output_Words,@fb1527d5@.UTIL.DNP_Server_Database.Binary_Output_Words) ] ,LES(@fb1527d5@.UTIL.DNP_Server_Database.Binary_Output_Words,@fb1527d5@.UTIL.DNP_Server_Database.PLC_Binary_Output_Words) COP(@fb1527d5@.UTIL.DNP_Server_Database.PLC_Binary_Output_Words,@fb1527d5@.UTIL.DNP_Server_Database.Binary_Output_Words,1) ,[XIO(@fb1527d5@.UTIL.DNP_Server_Database.Disable_Points.Disable_DNP_AO_16) SIZE(@fb1527d5@.DATA.DNP_Outputs.Analog16[0],0,@fb1527d5@.UTIL.DNP_Server_Database.PLC_Analog_Outputs) ,XIC(@fb1527d5@.UTIL.DNP_Server_Database.Disable_Points.Disable_DNP_AO_16) MOV(0,@fb1527d5@.UTIL.DNP_Server_Database.PLC_Analog_Outputs) ,XIO(@fb1527d5@.CONFIG.DNP3_Server.Use_Data_from_Client_connection) MOV(@fb1527d5@.UTIL.DNP_Server_Database.PLC_Analog_Outputs,@fb1527d5@.UTIL.DNP_Server_Database.Analog_Outputs) ] ,LES(@fb1527d5@.UTIL.DNP_Server_Database.Analog_Outputs,@fb1527d5@.UTIL.DNP_Server_Database.PLC_Analog_Outputs) COP(@fb1527d5@.UTIL.DNP_Server_Database.PLC_Analog_Outputs,@fb1527d5@.UTIL.DNP_Server_Database.Analog_Outputs,1) ,[XIO(@fb1527d5@.UTIL.DNP_Server_Database.Disable_Points.Disable_DNP_AO_32) SIZE(@fb1527d5@.DATA.DNP_Outputs.Analog32[0],0,@fb1527d5@.UTIL.DNP_Server_Database.PLC_Analog32_Outputs) ,XIC(@fb1527d5@.UTIL.DNP_Server_Database.Disable_Points.Disable_DNP_AO_32) MOV(0,@fb1527d5@.UTIL.DNP_Server_Database.PLC_Analog32_Outputs) ,XIO(@fb1527d5@.CONFIG.DNP3_Server.Use_Data_from_Client_connection) MOV(@fb1527d5@.UTIL.DNP_Server_Database.PLC_Analog32_Outputs,@fb1527d5@.UTIL.DNP_Server_Database.Analog32_Outputs) ] ,LES(@fb1527d5@.UTIL.DNP_Server_Database.Analog32_Outputs,@fb1527d5@.UTIL.DNP_Server_Database.PLC_Analog32_Outputs) COP(@fb1527d5@.UTIL.DNP_Server_Database.PLC_Analog32_Outputs,@fb1527d5@.UTIL.DNP_Server_Database.Analog32_Outputs,1) ,[XIO(@fb1527d5@.UTIL.DNP_Server_Database.Disable_Points.Disable_DNP_FO) SIZE(@fb1527d5@.DATA.DNP_Outputs.Float[0],0,@fb1527d5@.UTIL.DNP_Server_Database.PLC_Float_Outputs) ,XIC(@fb1527d5@.UTIL.DNP_Server_Database.Disable_Points.Disable_DNP_FO) MOV(0,@fb1527d5@.UTIL.DNP_Server_Database.PLC_Float_Outputs) ,XIO(@fb1527d5@.CONFIG.DNP3_Server.Use_Data_from_Client_connection) MOV(@fb1527d5@.UTIL.DNP_Server_Database.PLC_Float_Outputs,@fb1527d5@.UTIL.DNP_Server_Database.Float_Output) ] ,LES(@fb1527d5@.UTIL.DNP_Server_Database.Float_Output,@fb1527d5@.UTIL.DNP_Server_Database.PLC_Float_Outputs) COP(@fb1527d5@.UTIL.DNP_Server_Database.PLC_Float_Outputs,@fb1527d5@.UTIL.DNP_Server_Database.Float_Output,1) ,XIO(@fb1527d5@.CONFIG.DNP3_Server.Use_Double_Floats) [MOV(0,@fb1527d5@.UTIL.DNP_Server_Database.Double_Outputs) ,MOV(0,@fb1527d5@.UTIL.DNP_Server_Database.PLC_Double_Outputs) ] ,[XIC(@fb1527d5@.CONFIG.DNP3_Server.Use_Double_Floats) SIZE(@fb1527d5@.DATA.DNP_Outputs.Double[0],0,@fb1527d5@.UTIL.DNP_Server_Database.PLC_Double_Outputs) ,XIC(@fb1527d5@.CONFIG.DNP3_Server.Use_Double_Floats) XIO(@fb1527d5@.CONFIG.DNP3_Server.Use_Data_from_Client_connection) MOV(@fb1527d5@.UTIL.DNP_Server_Database.PLC_Double_Outputs,@fb1527d5@.UTIL.DNP_Server_Database.Double_Outputs) ] ,LES(@fb1527d5@.UTIL.DNP_Server_Database.Double_Outputs,@fb1527d5@.UTIL.DNP_Server_Database.PLC_Double_Outputs) COP(@fb1527d5@.UTIL.DNP_Server_Database.PLC_Double_Outputs,@fb1527d5@.UTIL.DNP_Server_Database.Double_Outputs,1) ,SIZE(@fb1527d5@.DATA.IED_Inputs.Binary[0],0,@fb1527d5@.UTIL.IED_Database.Binary_Input_Words) ,SIZE(@fb1527d5@.DATA.IED_Inputs.Analog16[0],0,@fb1527d5@.UTIL.IED_Database.Analog16_Inputs) ,SIZE(@fb1527d5@.DATA.IED_Inputs.Analog32[0],0,@fb1527d5@.UTIL.IED_Database.Analog32_Inputs) ,SIZE(@fb1527d5@.DATA.IED_Inputs.Float[0],0,@fb1527d5@.UTIL.IED_Database.Float_Inputs) ,SIZE(@fb1527d5@.DATA.IED_Inputs.Counter[0],0,@fb1527d5@.UTIL.IED_Database.Counters) ,SIZE(@fb1527d5@.DATA.IED_Outputs.Binary[0],0,@fb1527d5@.UTIL.IED_Database.Binary_Output_Words) ,SIZE(@fb1527d5@.DATA.IED_Outputs.Analog16[0],0,@fb1527d5@.UTIL.IED_Database.Analog16_Outputs) ,SIZE(@fb1527d5@.DATA.IED_Outputs.Analog32[0],0,@fb1527d5@.UTIL.IED_Database.Analog32_Outputs) ,SIZE(@fb1527d5@.DATA.IED_Outputs.Float[0],0,@fb1527d5@.UTIL.IED_Database.Float_Outputs) ,SIZE(@fb1527d5@.DATA.IED_Inputs.Binary_Out_Status[0],0,@fb1527d5@.UTIL.IED_Database.Binary_Out_Words_Status_Size) ,SIZE(@fb1527d5@.DATA.IED_Inputs.Analog16_Out_Status[0],0,@fb1527d5@.UTIL.IED_Database.Analog16_Out_Status_Size) ,SIZE(@fb1527d5@.DATA.IED_Inputs.Analog32_Out_Status[0],0,@fb1527d5@.UTIL.IED_Database.Analog32_Out_Status_Size) ,SIZE(@fb1527d5@.DATA.IED_Inputs.Float_Out_Status,0,@fb1527d5@.UTIL.IED_Database.Float_Out_Status_Size) ,OTU(@fb1527d5@.CONTROL.ChangeDatabaseSize) ];
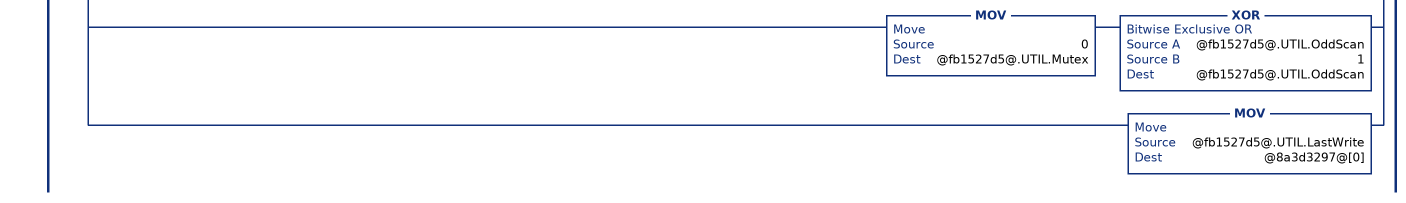
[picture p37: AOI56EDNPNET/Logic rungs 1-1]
   // This rung should only execute when the read data block from the DNPNET module is a NEW input data block.
   1: NEQ(@426a2124@[249],@fb1527d5@.UTIL.LastRead)[MOV(@426a2124@[249],@fb1527d5@.UTIL.LastRead) ,EQU(@fb1527d5@.UTIL.LastRead,1) [MOV(0,@fb1527d5@.UTIL.OffsetCounter) ,CPT(@fb1527d5@.UTIL.CopyLength,@fb1527d5@.UTIL.DNP_Server_Database.PLC_Binary_Output_Words) ,COP(@fb1527d5@.UTIL.ReadData[@fb1527d5@.UTIL.OffsetCounter],@fb1527d5@.DATA.DNP_Outputs.Binary[0],@fb1527d5@.UTIL.CopyLength) ,CPT(@fb1527d5@.UTIL.OffsetCounter,@fb1527d5@.UTIL.DNP_Server_Database.PLC_Binary_Output_Words) ,COP(@fb1527d5@.UTIL.ReadData[@fb1527d5@.UTIL.OffsetCounter],@fb1527d5@.DATA.DNP_Outputs.Analog16[0],@fb1527d5@.UTIL.DNP_Server_Database.PLC_Analog_Outputs) ,CPT(@fb1527d5@.UTIL.OffsetCounter,@fb1527d5@.UTIL.DNP_Server_Database.PLC_Analog_Outputs+@fb1527d5@.UTIL.OffsetCounter) ,COP(@fb1527d5@.UTIL.ReadData[@fb1527d5@.UTIL.OffsetCounter],@fb1527d5@.DATA.DNP_Outputs.Analog32[0],@fb1527d5@.UTIL.DNP_Server_Database.PLC_Analog32_Outputs) ,CPT(@fb1527d5@.UTIL.OffsetCounter,2*@fb1527d5@.UTIL.DNP_Server_Database.PLC_Analog32_Outputs+@fb1527d5@.UTIL.OffsetCounter) ,COP(@fb1527d5@.UTIL.ReadData[@fb1527d5@.UTIL.OffsetCounter],@fb1527d5@.DATA.DNP_Outputs.Float[0],@fb1527d5@.UTIL.DNP_Server_Database.PLC_Float_Outputs) ,CPT(@fb1527d5@.UTIL.OffsetCounter,2*@fb1527d5@.UTIL.DNP_Server_Database.PLC_Float_Outputs+@fb1527d5@.UTIL.OffsetCounter) ,COP(@fb1527d5@.UTIL.ReadData[@fb1527d5@.UTIL.OffsetCounter],@fb1527d5@.DATA.DNP_Outputs.Double[0],@fb1527d5@.UTIL.DNP_Server_Database.PLC_Double_Outputs) ,CPT(@fb1527d5@.UTIL.OffsetCounter,4*@fb1527d5@.UTIL.DNP_Server_Database.PLC_Double_Outputs+@fb1527d5@.UTIL.OffsetCounter) ,CPT(@fb1527d5@.UTIL.CopyLength,@fb1527d5@.UTIL.IED_Database.Binary_Input_Words) ,COP(@fb1527d5@.UTIL.ReadData[@fb1527d5@.UTIL.OffsetCounter],@fb1527d5@.DATA.IED_Inputs.Binary[0],@fb1527d5@.UTIL.CopyLength) ,CPT(@fb1527d5@.UTIL.OffsetCounter,@fb1527d5@.UTIL.IED_Database.Binary_Input_Words+@fb1527d5@.UTIL.OffsetCounter) ,COP(@fb1527d5@.UTIL.ReadData[@fb1527d5@.UTIL.OffsetCounter],@fb1527d5@.DATA.IED_Inputs.Analog16[0],@fb1527d5@.UTIL.IED_Database.Analog16_Inputs) ,CPT(@fb1527d5@.UTIL.OffsetCounter,@fb1527d5@.UTIL.IED_Database.Analog16_Inputs+@fb1527d5@.UTIL.OffsetCounter) ,COP(@fb1527d5@.UTIL.ReadData[@fb1527d5@.UTIL.OffsetCounter],@fb1527d5@.DATA.IED_Inputs.Analog32[0],@fb1527d5@.UTIL.IED_Database.Analog32_Inputs) ,CPT(@fb1527d5@.UTIL.OffsetCounter,2*@fb1527d5@.UTIL.IED_Database.Analog32_Inputs+@fb1527d5@.UTIL.OffsetCounter) ,COP(@fb1527d5@.UTIL.ReadData[@fb1527d5@.UTIL.OffsetCounter],@fb1527d5@.DATA.IED_Inputs.Float[0],@fb1527d5@.UTIL.IED_Database.Float_Inputs) ,CPT(@fb1527d5@.UTIL.OffsetCounter,2*@fb1527d5@.UTIL.IED_Database.Float_Inputs+@fb1527d5@.UTIL.OffsetCounter) ,COP(@fb1527d5@.UTIL.ReadData[@fb1527d5@.UTIL.OffsetCounter],@fb1527d5@.DATA.IED_Inputs.Counter[0],@fb1527d5@.UTIL.IED_Database.Counters) ,CPT(@fb1527d5@.UTIL.OffsetCounter,2*@fb1527d5@.UTIL.IED_Database.Counters+@fb1527d5@.UTIL.OffsetCounter) ,EQU(@fb1527d5@.CONFIG.DNP3_Client.Use_Binary_Output_status_Data,1) COP(@fb1527d5@.UTIL.ReadData[@fb1527d5@.UTIL.OffsetCounter],@fb1527d5@.DATA.IED_Inputs.Binary_Out_Status[0],@fb1527d5@.UTIL.IED_Database.Binary_Out_Words_Status_Size) ,EQU(@fb1527d5@.CONFIG.DNP3_Client.Use_Analog_Output_status_Data,1) [CPT(@fb1527d5@.UTIL.OffsetCounter,@fb1527d5@.UTIL.IED_Database.Binary_Out_Words_Status_Size+@fb1527d5@.UTIL.OffsetCounter) ,COP(@fb1527d5@.UTIL.ReadData[@fb1527d5@.UTIL.OffsetCounter],@fb1527d5@.DATA.IED_Inputs.Analog16_Out_Status[0],@fb1527d5@.UTIL.IED_Database.Analog16_Out_Status_Size) ,CPT(@fb1527d5@.UTIL.OffsetCounter,@fb1527d5@.UTIL.IED_Database.Analog16_Out_Status_Size+@fb1527d5@.UTIL.OffsetCounter) ,COP(@fb1527d5@.UTIL.ReadData[@fb1527d5@.UTIL.OffsetCounter],@fb1527d5@.DATA.IED_Inputs.Analog32_Out_Status[0],@fb1527d5@.UTIL.IED_Database.Analog32_Out_Status_Size) ,CPT(@fb1527d5@.UTIL.OffsetCounter,2*@fb1527d5@.UTIL.IED_Database.Analog32_Out_Status_Size+@fb1527d5@.UTIL.OffsetCounter) ,COP(@fb1527d5@.UTIL.ReadData[@fb1527d5@.UTIL.OffsetCounter],@fb1527d5@.DATA.IED_Inputs.Float_Out_Status[0],@fb1527d5@.UTIL.IED_Database.Float_Out_Status_Size) ] ] ,LIM(1,@fb1527d5@.UTIL.LastRead,203) [CPT(@fb1527d5@.UTIL.BlockIndex,(@fb1527d5@.UTIL.LastRead-1)*240) ,COP(@426a2124@[2],@fb1527d5@.UTIL.ReadData[@fb1527d5@.UTIL.BlockIndex],240) ] ,EQU(@fb1527d5@.UTIL.LastRead,300) [COP(@426a2124@[2],@fb1527d5@.STATUS.GenStat.Cur_Port,70) ,COP(@426a2124@[80],@fb1527d5@.STATUS.ErrorList[0],60) ,COP(@426a2124@[140],@fb1527d5@.STATUS.IINServerBits[0],40) ,COP(@426a2124@[180],@fb1527d5@.STATUS.Network.TCP_Parsing,17) ] ,EQU(@fb1527d5@.UTIL.LastRead,9902) [MOV(@426a2124@[2],@fb1527d5@.CONTROL.CommandControl.NumberofCommands) ,OTU(@fb1527d5@.CONTROL.CommandControl.Send) ] ,EQU(@fb1527d5@.UTIL.LastRead,9903) [MOV(@426a2124@[2],@fb1527d5@.CONTROL.Events.CountPerBlock) ,COP(@426a2124@[3],@fb1527d5@.CONTROL.EventMessages[0].Device_Index,240) ,MOV(@426a2124@[243],@fb1527d5@.CONTROL.Events.BufferOverflow) ,MOV(@426a2124@[244],@fb1527d5@.CONTROL.Events.Queued) ,ONS(@fb1527d5@.CONTROL.Events.OneShot) [EQU(@fb1527d5@.CONTROL.Events.BlockTransferCount,0) MOV(0,@fb1527d5@.CONTROL.Events.CountTotal) ,[ADD(@fb1527d5@.CONTROL.Events.CountPerBlock,@fb1527d5@.CONTROL.Events.CountTotal,@fb1527d5@.CONTROL.Events.CountTotal) ,ADD(@fb1527d5@.CONTROL.Events.CountPerBlock,@fb1527d5@.CONTROL.Events.CEC,@fb1527d5@.CONTROL.Events.CEC) ,GRT(@fb1527d5@.CONTROL.Events.CEC,2147483631) SUB(@fb1527d5@.CONTROL.Events.CEC,2147483631,@fb1527d5@.CONTROL.Events.CEC) ] ,ADD(1,@fb1527d5@.CONTROL.Events.BlockTransferCount,@fb1527d5@.CONTROL.Events.BlockTransferCount) ,EQU(@fb1527d5@.CONTROL.Events.Queued,0) [MOV(@fb1527d5@.CONTROL.Events.BlockTransferCount,@fb1527d5@.CONTROL.Events.BTCountTotal) ,MOV(0,@fb1527d5@.CONTROL.Events.BlockTransferCount) ] ,ADD(1,@fb1527d5@.CONTROL.Events.CBC,@fb1527d5@.CONTROL.Events.CBC) ,EQU(@fb1527d5@.CONTROL.Events.CBC,2147483646) MOV(0,@fb1527d5@.CONTROL.Events.CBC) ] ] ,EQU(@fb1527d5@.UTIL.LastRead,9910) [MOV(@426a2124@[2],@fb1527d5@.CONTROL.CROBmsg_counter.CountPerBlock) ,COP(@426a2124@[3],@fb1527d5@.CONTROL.CROBmsg_data[0].Point_Number,240) ,ONS(@fb1527d5@.CONTROL.CROBmsg_counter.OneShot) [ADD(@fb1527d5@.CONTROL.CROBmsg_counter.CountPerBlock,@fb1527d5@.CONTROL.CROBmsg_counter.CCC,@fb1527d5@.CONTROL.CROBmsg_counter.CCC) ,GRT(@fb1527d5@.CONTROL.CROBmsg_counter.CCC,2147483606) SUB(@fb1527d5@.CONTROL.CROBmsg_counter.CCC,2147483606,@fb1527d5@.CONTROL.CROBmsg_counter.CCC) ,ADD(1,@fb1527d5@.CONTROL.CROBmsg_counter.CCBC,@fb1527d5@.CONTROL.CROBmsg_counter.CCBC) ,EQU(@fb1527d5@.CONTROL.CROBmsg_counter.CCBC,2147483646) MOV(0,@fb1527d5@.CONTROL.CROBmsg_counter.CCBC) ] ] ,EQU(@fb1527d5@.UTIL.LastRead,9949) [MOV(@426a2124@[2],@fb1527d5@.UTIL.CopyLength) ,MOV(@426a2124@[3],@fb1527d5@.UTIL.OffsetCounter) ,CPT(@fb1527d5@.UTIL.CopyLength,8 * @fb1527d5@.UTIL.CopyLength) ,COP(@426a2124@[4],@fb1527d5@.STATUS.ServerCommErrors[@fb1527d5@.UTIL.OffsetCounter],@fb1527d5@.UTIL.CopyLength) ,OTU(@fb1527d5@.CONTROL.Server_Comm_Errors.Request) ] ,EQU(@fb1527d5@.UTIL.LastRead,9950) [MOV(@426a2124@[3],@fb1527d5@.UTIL.OffsetCounter) ,COP(@426a2124@[4],@fb1527d5@.STATUS.CommandErrors[@fb1527d5@.UTIL.OffsetCounter],@426a2124@[2]) ,OTU(@fb1527d5@.CONTROL.Command_Errors.Request) ] ,EQU(@fb1527d5@.UTIL.LastRead,9958) [COP(@426a2124@[2],@fb1527d5@.CONTROL.Binary_Event_CalTime.Event_Count_Rec,2) ,OTU(@fb1527d5@.CONTROL.Binary_Event_CalTime.Send) ] ,EQU(@fb1527d5@.UTIL.LastRead,9959) [COP(@426a2124@[2],@fb1527d5@.CONTROL.Analog_Event_CalTime.Event_Count_Rec,2) ,OTU(@fb1527d5@.CONTROL.Analog_Event_CalTime.Send) ] ,EQU(@fb1527d5@.UTIL.LastRead,9968) [COP(@426a2124@[2],@fb1527d5@.CONTROL.Binary_Event_CLXTime.Event_Count_Rec,2) ,OTU(@fb1527d5@.CONTROL.Binary_Event_CLXTime.Send) ] ,EQU(@fb1527d5@.UTIL.LastRead,9969) [COP(@426a2124@[2],@fb1527d5@.CONTROL.Analog_Event_CLXTime.Event_Count_Rec,2) ,OTU(@fb1527d5@.CONTROL.Analog_Event_CLXTime.Send) ] ,EQU(@fb1527d5@.UTIL.LastRead,9970) XIC(@fb1527d5@.CONTROL.Get_Module_Time.Request) [MOV(@426a2124@[2],@fb1527d5@.CONTROL.Get_Module_Time.Clock.Year) ,MOV(@426a2124@[3],@fb1527d5@.CONTROL.Get_Module_Time.Clock.Month) ,MOV(@426a2124@[4],@fb1527d5@.CONTROL.Get_Module_Time.Clock.Day) ,MOV(@426a2124@[5],@fb1527d5@.CONTROL.Get_Module_Time.Clock.Hours) ,MOV(@426a2124@[6],@fb1527d5@.CONTROL.Get_Module_Time.Clock.Minutes) ,MOV(@426a2124@[7],@fb1527d5@.CONTROL.Get_Module_Time.Clock.Seconds) ,MUL(@426a2124@[8],1000,@fb1527d5@.CONTROL.Get_Module_Time.Clock.MicroSeconds) ,MOV(@426a2124@[9],@fb1527d5@.CONTROL.Get_Module_Time.Clock.Synchronized) ,XIC(@fb1527d5@.CONTROL.Get_Module_Time.Set_PLC_Time) EQU(@fb1527d5@.CONTROL.Get_Module_Time.Clock.Synchronized,1) [SSV(WallClockTime,,DateTime,@fb1527d5@.CONTROL.Get_Module_Time.Clock.Year) ,OTU(@fb1527d5@.CONTROL.Get_Module_Time.Set_PLC_Time) ] ,OTU(@fb1527d5@.CONTROL.Get_Module_Time.Request) ] ,MOV(@426a2124@[1],@fb1527d5@.UTIL.LastWrite) ,EQU(@fb1527d5@.UTIL.LastWrite,1) [CPT(@fb1527d5@.UTIL.OffsetCounter,0) ,CPT(@fb1527d5@.UTIL.CopyLength,@fb1527d5@.UTIL.DNP_Server_Database.PLC_Binary_Input_Words) ,COP(@fb1527d5@.DATA.DNP_Inputs.Binary[0],@fb1527d5@.UTIL.WriteData[@fb1527d5@.UTIL.OffsetCounter],@fb1527d5@.UTIL.CopyLength) ,CPT(@fb1527d5@.UTIL.OffsetCounter,@fb1527d5@.UTIL.CopyLength+@fb1527d5@.UTIL.OffsetCounter) ,CPT(@fb1527d5@.UTIL.CopyLength,@fb1527d5@.UTIL.DNP_Server_Database.PLC_Analog_Inputs) ,COP(@fb1527d5@.DATA.DNP_Inputs.Analog16[0],@fb1527d5@.UTIL.WriteData[@fb1527d5@.UTIL.OffsetCounter],@fb1527d5@.UTIL.CopyLength) ,CPT(@fb1527d5@.UTIL.OffsetCounter,@fb1527d5@.UTIL.CopyLength+@fb1527d5@.UTIL.OffsetCounter) ,CPT(@fb1527d5@.UTIL.CopyLength,@fb1527d5@.UTIL.DNP_Server_Database.PLC_Analog32_Inputs*2) ,COP(@fb1527d5@.DATA.DNP_Inputs.Analog32[0],@fb1527d5@.UTIL.WriteData[@fb1527d5@.UTIL.OffsetCounter],@fb1527d5@.UTIL.CopyLength) ,CPT(@fb1527d5@.UTIL.OffsetCounter,@fb1527d5@.UTIL.CopyLength+@fb1527d5@.UTIL.OffsetCounter) ,CPT(@fb1527d5@.UTIL.CopyLength,@fb1527d5@.UTIL.DNP_Server_Database.PLC_Float_Inputs*2) ,COP(@fb1527d5@.DATA.DNP_Inputs.Float[0],@fb1527d5@.UTIL.WriteData[@fb1527d5@.UTIL.OffsetCounter],@fb1527d5@.UTIL.CopyLength) ,CPT(@fb1527d5@.UTIL.OffsetCounter,@fb1527d5@.UTIL.CopyLength+@fb1527d5@.UTIL.OffsetCounter) ,CPT(@fb1527d5@.UTIL.CopyLength,@fb1527d5@.UTIL.DNP_Server_Database.PLC_Double_Inputs*4) ,COP(@fb1527d5@.DATA.DNP_Inputs.Double[0],@fb1527d5@.UTIL.WriteData[@fb1527d5@.UTIL.OffsetCounter],@fb1527d5@.UTIL.CopyLength) ,CPT(@fb1527d5@.UTIL.OffsetCounter,@fb1527d5@.UTIL.CopyLength+@fb1527d5@.UTIL.OffsetCounter) ,CPT(@fb1527d5@.UTIL.CopyLength,@fb1527d5@.UTIL.DNP_Server_Database.PLC_Counters*2) ,COP(@fb1527d5@.DATA.DNP_Inputs.Counter[0],@fb1527d5@.UTIL.WriteData[@fb1527d5@.UTIL.OffsetCounter],@fb1527d5@.UTIL.CopyLength) ,CPT(@fb1527d5@.UTIL.OffsetCounter,@fb1527d5@.UTIL.CopyLength+@fb1527d5@.UTIL.OffsetCounter) ,CPT(@fb1527d5@.UTIL.CopyLength,@fb1527d5@.UTIL.IED_Database.Binary_Output_Words) ,COP(@fb1527d5@.DATA.IED_Outputs.Binary[0],@fb1527d5@.UTIL.WriteData[@fb1527d5@.UTIL.OffsetCounter],@fb1527d5@.UTIL.CopyLength) ,CPT(@fb1527d5@.UTIL.OffsetCounter,@fb1527d5@.UTIL.CopyLength+@fb1527d5@.UTIL.OffsetCounter) ,CPT(@fb1527d5@.UTIL.CopyLength,@fb1527d5@.UTIL.IED_Database.Analog16_Outputs) ,COP(@fb1527d5@.DATA.IED_Outputs.Analog16[0],@fb1527d5@.UTIL.WriteData[@fb1527d5@.UTIL.OffsetCounter],@fb1527d5@.UTIL.CopyLength) ,CPT(@fb1527d5@.UTIL.OffsetCounter,@fb1527d5@.UTIL.CopyLength+@fb1527d5@.UTIL.OffsetCounter) ,CPT(@fb1527d5@.UTIL.CopyLength,@fb1527d5@.UTIL.IED_Database.Analog32_Outputs*2) ,COP(@fb1527d5@.DATA.IED_Outputs.Analog32[0],@fb1527d5@.UTIL.WriteData[@fb1527d5@.UTIL.OffsetCounter],@fb1527d5@.UTIL.CopyLength) ,CPT(@fb1527d5@.UTIL.OffsetCounter,@fb1527d5@.UTIL.CopyLength+@fb1527d5@.UTIL.OffsetCounter) ,CPT(@fb1527d5@.UTIL.CopyLength,@fb1527d5@.UTIL.IED_Database.Float_Outputs*2) ,COP(@fb1527d5@.DATA.IED_Outputs.Float[0],@fb1527d5@.UTIL.WriteData[@fb1527d5@.UTIL.OffsetCounter],@fb1527d5@.UTIL.CopyLength) ] ,LIM(1,@fb1527d5@.UTIL.LastWrite,117) [CPT(@fb1527d5@.UTIL.BlockIndex,(@fb1527d5@.UTIL.LastWrite - 1) * 240) ,COP(@fb1527d5@.UTIL.WriteData[@fb1527d5@.UTIL.BlockIndex],@8a3d3297@[1],240) ] ,LIM(1000,@fb1527d5@.UTIL.LastWrite,1022) [CPT(@fb1527d5@.UTIL.BlockIndex,(@fb1527d5@.UTIL.LastWrite - 1000) * 240) ,COP(@fb1527d5@.UTIL.ReadData[@fb1527d5@.UTIL.BlockIndex],@8a3d3297@[1],240) ,MOV(1,@fb1527d5@.UTIL.Mutex) ] ,LIM(1100,@fb1527d5@.UTIL.LastWrite,1193) [CPT(@fb1527d5@.UTIL.OffsetCounter,@fb1527d5@.UTIL.DNP_Server_Database.PLC_Binary_Output_Words) ,CPT(@fb1527d5@.UTIL.OffsetCounter,@fb1527d5@.UTIL.OffsetCounter + @fb1527d5@.UTIL.DNP_Server_Database.PLC_Analog_Outputs) ,CPT(@fb1527d5@.UTIL.OffsetCounter,@fb1527d5@.UTIL.OffsetCounter + (2 * @fb1527d5@.UTIL.DNP_Server_Database.PLC_Analog32_Outputs)) ,CPT(@fb1527d5@.UTIL.OffsetCounter,@fb1527d5@.UTIL.OffsetCounter + (2 * @fb1527d5@.UTIL.DNP_Server_Database.PLC_Float_Outputs)) ,CPT(@fb1527d5@.UTIL.OffsetCounter,@fb1527d5@.UTIL.OffsetCounter + (4 * @fb1527d5@.UTIL.DNP_Server_Database.PLC_Double_Outputs)) ,CPT(@fb1527d5@.UTIL.BlockIndex,@fb1527d5@.UTIL.OffsetCounter + ((@fb1527d5@.UTIL.LastWrite - 1100) * 240)) ,COP(@fb1527d5@.UTIL.ReadData[@fb1527d5@.UTIL.BlockIndex],@8a3d3297@[1],240) ,MOV(1,@fb1527d5@.UTIL.Mutex) ] ,EQU(@fb1527d5@.UTIL.LastWrite,9000) [SIZE(@fb1527d5@.CONFIG.DNP_Server_Override.Binary_Inputs[0],0,@fb1527d5@.UTIL.DNP_List_Entry_Counts.BI_Class_Overrides) ,SIZE(@fb1527d5@.CONFIG.DNP_Server_Override.Analog16_Inputs[0],0,@fb1527d5@.UTIL.DNP_List_Entry_Counts.AI_ClassDeadband_Overrides) ,SIZE(@fb1527d5@.CONFIG.DNP_Server_Override.Analog32_Inputs[0],0,@fb1527d5@.UTIL.DNP_List_Entry_Counts.A32I_ClassDeadband_Overrides) ,SIZE(@fb1527d5@.CONFIG.DNP_Server_Override.Float_Inputs[0],0,@fb1527d5@.UTIL.DNP_List_Entry_Counts.FLTI_ClassDeadband_Overrides) ,SIZE(@fb1527d5@.CONFIG.DNP_Server_Override.Double_Inputs[0],0,@fb1527d5@.UTIL.DNP_List_Entry_Counts.DBLI_ClassDeadband_Overrides) ,SIZE(@fb1527d5@.CONFIG.DNP_Server_List[0],0,@fb1527d5@.UTIL.DNP_List_Entry_Counts.Server_List_Entries) ,SIZE(@fb1527d5@.CONFIG.DNP_Client_Commands[0],0,@fb1527d5@.UTIL.DNP_List_Entry_Counts.Client_Commands) ,COP(@fb1527d5@.CONFIG.DNP_Module_Name[0],@8a3d3297@[1],20) ,COP(@fb1527d5@.CONFIG.DNP3_Server.Internal_Server_ID,@8a3d3297@[21],36) ,COP(@fb1527d5@.CONFIG.DNP3_WhiteList[0].a,@8a3d3297@[57],40) ,COP(@fb1527d5@.UTIL.DNP_Server_Database.Binary_Input_Words,@8a3d3297@[97],22) ,COP(@fb1527d5@.CONFIG.DNP3_Client.Internal_ID,@8a3d3297@[119],8) ,COP(@fb1527d5@.UTIL.IED_Database.Binary_Input_Words,@8a3d3297@[127],10) ,COP(@fb1527d5@.UTIL.DNP_List_Entry_Counts.BI_Class_Overrides,@8a3d3297@[137],8) ,MOV(1,@fb1527d5@.UTIL.Mutex) ] ,LIM(9001,@fb1527d5@.UTIL.LastWrite,9099) [MOV(0,@fb1527d5@.UTIL.OffsetCounter) ,CPT(@fb1527d5@.UTIL.CopyLength,2*@fb1527d5@.UTIL.DNP_List_Entry_Counts.BI_Class_Overrides) ,COP(@fb1527d5@.CONFIG.DNP_Server_Override.Binary_Inputs[0],@fb1527d5@.UTIL.WriteData[@fb1527d5@.UTIL.OffsetCounter],@fb1527d5@.UTIL.CopyLength) ,CPT(@fb1527d5@.UTIL.OffsetCounter,@fb1527d5@.UTIL.CopyLength + @fb1527d5@.UTIL.OffsetCounter) ,CPT(@fb1527d5@.UTIL.CopyLength,4*@fb1527d5@.UTIL.DNP_List_Entry_Counts.AI_ClassDeadband_Overrides) ,COP(@fb1527d5@.CONFIG.DNP_Server_Override.Analog16_Inputs[0],@fb1527d5@.UTIL.WriteData[@fb1527d5@.UTIL.OffsetCounter],@fb1527d5@.UTIL.CopyLength) ,CPT(@fb1527d5@.UTIL.OffsetCounter,@fb1527d5@.UTIL.CopyLength + @fb1527d5@.UTIL.OffsetCounter) ,CPT(@fb1527d5@.UTIL.CopyLength,4*@fb1527d5@.UTIL.DNP_List_Entry_Counts.A32I_ClassDeadband_Overrides) ,COP(@fb1527d5@.CONFIG.DNP_Server_Override.Analog32_Inputs[0],@fb1527d5@.UTIL.WriteData[@fb1527d5@.UTIL.OffsetCounter],@fb1527d5@.UTIL.CopyLength) ,CPT(@fb1527d5@.UTIL.OffsetCounter,@fb1527d5@.UTIL.CopyLength + @fb1527d5@.UTIL.OffsetCounter) ,CPT(@fb1527d5@.UTIL.CopyLength,4*@fb1527d5@.UTIL.DNP_List_Entry_Counts.FLTI_ClassDeadband_Overrides) ,COP(@fb1527d5@.CONFIG.DNP_Server_Override.Float_Inputs[0],@fb1527d5@.UTIL.WriteData[@fb1527d5@.UTIL.OffsetCounter],@fb1527d5@.UTIL.CopyLength) ,CPT(@fb1527d5@.UTIL.OffsetCounter,@fb1527d5@.UTIL.CopyLength + @fb1527d5@.UTIL.OffsetCounter) ,CPT(@fb1527d5@.UTIL.CopyLength,4*@fb1527d5@.UTIL.DNP_List_Entry_Counts.DBLI_ClassDeadband_Overrides) ,COP(@fb1527d5@.CONFIG.DNP_Server_Override.Double_Inputs[0],@fb1527d5@.UTIL.WriteData[@fb1527d5@.UTIL.OffsetCounter],@fb1527d5@.UTIL.CopyLength) ,CPT(@fb1527d5@.UTIL.OffsetCounter,@fb1527d5@.UTIL.CopyLength+@fb1527d5@.UTIL.OffsetCounter) ,CPT(@fb1527d5@.UTIL.CopyLength,14*@fb1527d5@.UTIL.DNP_List_Entry_Counts.Server_List_Entries) ,COP(@fb1527d5@.CONFIG.DNP_Server_List[0],@fb1527d5@.UTIL.WriteData[@fb1527d5@.UTIL.OffsetCounter],@fb1527d5@.UTIL.CopyLength) ,CPT(@fb1527d5@.UTIL.OffsetCounter,@fb1527d5@.UTIL.CopyLength + @fb1527d5@.UTIL.OffsetCounter) ,CPT(@fb1527d5@.UTIL.CopyLength,10*@fb1527d5@.UTIL.DNP_List_Entry_Counts.Client_Commands) ,COP(@fb1527d5@.CONFIG.DNP_Client_Commands[0],@fb1527d5@.UTIL.WriteData[@fb1527d5@.UTIL.OffsetCounter],@fb1527d5@.UTIL.CopyLength) ,CPT(@fb1527d5@.UTIL.BlockIndex,(@fb1527d5@.UTIL.LastWrite - 9001) * 240) ,COP(@fb1527d5@.UTIL.WriteData[@fb1527d5@.UTIL.BlockIndex],@8a3d3297@[1],240) ,MOV(1,@fb1527d5@.UTIL.Mutex) ] ,XIC(@fb1527d5@.CONTROL.CROB_Commands.Send) EQU(@fb1527d5@.UTIL.OddScan,0) EQU(@fb1527d5@.UTIL.Mutex,0) LES(@fb1527d5@.UTIL.LastService,9901) [COP(@fb1527d5@.CONTROL.CROB_Commands.Command_Count,@8a3d3297@[1],1) ,COP(@fb1527d5@.CONTROL.CROB_Commands.CROB_Commands[0],@8a3d3297@[2],240) ,MOV(9901,@fb1527d5@.UTIL.LastService) ,MOV(1,@fb1527d5@.UTIL.Mutex) ,MOV(9901,@fb1527d5@.UTIL.LastWrite) ,OTU(@fb1527d5@.CONTROL.CROB_Commands.Send) ] ,XIC(@fb1527d5@.CONTROL.CommandControl.Send) EQU(@fb1527d5@.UTIL.OddScan,0) EQU(@fb1527d5@.UTIL.Mutex,0) LES(@fb1527d5@.UTIL.LastService,9902) [COP(@fb1527d5@.CONTROL.CommandControl.NumberofCommands,@8a3d3297@[1],1) ,COP(@fb1527d5@.CONTROL.CommandControl.ClientCommands[0],@8a3d3297@[2],240) ,MOV(9902,@fb1527d5@.UTIL.LastService) ,MOV(1,@fb1527d5@.UTIL.Mutex) ,MOV(9902,@fb1527d5@.UTIL.LastWrite) ] ,XIC(@fb1527d5@.CONTROL.Aux_Commands.Send) EQU(@fb1527d5@.UTIL.OddScan,0) EQU(@fb1527d5@.UTIL.Mutex,0) LES(@fb1527d5@.UTIL.LastService,9904) [COP(@fb1527d5@.CONTROL.Aux_Commands.Command_Count,@8a3d3297@[1],1) ,COP(@fb1527d5@.CONTROL.Aux_Commands.Commands[0],@8a3d3297@[2],240) ,MOV(9904,@fb1527d5@.UTIL.LastService) ,MOV(1,@fb1527d5@.UTIL.Mutex) ,MOV(9904,@fb1527d5@.UTIL.LastWrite) ,OTU(@fb1527d5@.CONTROL.Aux_Commands.Send) ] ,XIC(@fb1527d5@.CONTROL.Server_Comm_Errors.Request) EQU(@fb1527d5@.UTIL.OddScan,0) EQU(@fb1527d5@.UTIL.Mutex,0) LES(@fb1527d5@.UTIL.LastService,9949) [COP(@fb1527d5@.CONTROL.Server_Comm_Errors.Number_of_Servers,@8a3d3297@[1],2) ,MOV(9949,@fb1527d5@.UTIL.LastService) ,MOV(1,@fb1527d5@.UTIL.Mutex) ,MOV(9949,@fb1527d5@.UTIL.LastWrite) ] ,XIC(@fb1527d5@.CONTROL.Command_Errors.Request) EQU(@fb1527d5@.UTIL.OddScan,0) EQU(@fb1527d5@.UTIL.Mutex,0) LES(@fb1527d5@.UTIL.LastService,9950) [COP(@fb1527d5@.CONTROL.Command_Errors.Number_Of_Commands,@8a3d3297@[1],2) ,MOV(9950,@fb1527d5@.UTIL.LastService) ,MOV(1,@fb1527d5@.UTIL.Mutex) ,MOV(9950,@fb1527d5@.UTIL.LastWrite) ] ,XIC(@fb1527d5@.CONTROL.Binary_Event_CalTime.Send) EQU(@fb1527d5@.UTIL.OddScan,0) EQU(@fb1527d5@.UTIL.Mutex,0) LES(@fb1527d5@.UTIL.LastService,9958) [COP(@fb1527d5@.CONTROL.Binary_Event_CalTime.Event_Count,@8a3d3297@[1],2) ,COP(@fb1527d5@.CONTROL.Binary_Event_CalTime.Event[0].Point_Number,@8a3d3297@[3],240) ,MOV(9958,@fb1527d5@.UTIL.LastService) ,MOV(1,@fb1527d5@.UTIL.Mutex) ,MOV(9958,@fb1527d5@.UTIL.LastWrite) ] ,XIC(@fb1527d5@.CONTROL.Analog_Event_CalTime.Send) EQU(@fb1527d5@.UTIL.OddScan,0) EQU(@fb1527d5@.UTIL.Mutex,0) LES(@fb1527d5@.UTIL.LastService,9959) [COP(@fb1527d5@.CONTROL.Analog_Event_CalTime.Event_Count,@8a3d3297@[1],2) ,COP(@fb1527d5@.CONTROL.Analog_Event_CalTime.Event[0].Point_Number,@8a3d3297@[3],240) ,MOV(9959,@fb1527d5@.UTIL.LastService) ,MOV(1,@fb1527d5@.UTIL.Mutex) ,MOV(9959,@fb1527d5@.UTIL.LastWrite) ] ,XIC(@fb1527d5@.CONTROL.Binary_Event_CLXTime.Send) EQU(@fb1527d5@.UTIL.OddScan,0) EQU(@fb1527d5@.UTIL.Mutex,0) LES(@fb1527d5@.UTIL.LastService,9968) [COP(@fb1527d5@.CONTROL.Binary_Event_CLXTime.Event_Count,@8a3d3297@[1],2) ,COP(@fb1527d5@.CONTROL.Binary_Event_CLXTime.Event[0].Point_Number,@8a3d3297@[3],240) ,MOV(9968,@fb1527d5@.UTIL.LastService) ,MOV(1,@fb1527d5@.UTIL.Mutex) ,MOV(9968,@fb1527d5@.UTIL.LastWrite) ] ,XIC(@fb1527d5@.CONTROL.Analog_Event_CLXTime.Send) EQU(@fb1527d5@.UTIL.OddScan,0) EQU(@fb1527d5@.UTIL.Mutex,0) LES(@fb1527d5@.UTIL.LastService,9969) [COP(@fb1527d5@.CONTROL.Analog_Event_CLXTime.Event_Count,@8a3d3297@[1],2) ,COP(@fb1527d5@.CONTROL.Analog_Event_CLXTime.Event[0].Point_Number,@8a3d3297@[3],240) ,MOV(9969,@fb1527d5@.UTIL.LastService) ,MOV(1,@fb1527d5@.UTIL.Mutex) ,MOV(9969,@fb1527d5@.UTIL.LastWrite) ] ,XIC(@fb1527d5@.CONTROL.Get_Module_Time.Request) EQU(@fb1527d5@.UTIL.OddScan,0) EQU(@fb1527d5@.UTIL.Mutex,0) LES(@fb1527d5@.UTIL.LastService,9970) [MOV(9970,@fb1527d5@.UTIL.LastService) ,MOV(1,@fb1527d5@.UTIL.Mutex) ,MOV(9970,@fb1527d5@.UTIL.LastWrite) ] ,XIC(@fb1527d5@.CONTROL.Set_Module_Time.Send) EQU(@fb1527d5@.UTIL.OddScan,0) EQU(@fb1527d5@.UTIL.Mutex,0) LES(@fb1527d5@.UTIL.LastService,9971) [GSV(WallClockTime,,DateTime,@fb1527d5@.CONTROL.Set_Module_Time.PLC_Time[0]) ,MOV(@fb1527d5@.CONTROL.Set_Module_Time.PLC_Time[0],@8a3d3297@[1]) ,MOV(@fb1527d5@.CONTROL.Set_Module_Time.PLC_Time[1],@8a3d3297@[2]) ,MOV(@fb1527d5@.CONTROL.Set_Module_Time.PLC_Time[2],@8a3d3297@[3]) ,MOV(@fb1527d5@.CONTROL.Set_Module_Time.PLC_Time[3],@8a3d3297@[4]) ,MOV(@fb1527d5@.CONTROL.Set_Module_Time.PLC_Time[4],@8a3d3297@[5]) ,MOV(@fb1527d5@.CONTROL.Set_Module_Time.PLC_Time[5],@8a3d3297@[6]) ,DIV(@fb1527d5@.CONTROL.Set_Module_Time.PLC_Time[6],100,@8a3d3297@[7]) ,MOV(9971,@fb1527d5@.UTIL.LastService) ,MOV(1,@fb1527d5@.UTIL.Mutex) ,MOV(9971,@fb1527d5@.UTIL.LastWrite) ,OTU(@fb1527d5@.CONTROL.Set_Module_Time.Send) ] ,XIC(@fb1527d5@.CONTROL.WarmBoot) [MOV(9998,@fb1527d5@.UTIL.LastWrite) ,EQU(@8a3d3297@[0],9998) OTU(@fb1527d5@.CONTROL.WarmBoot) ] ,XIC(@fb1527d5@.CONTROL.ColdBoot) [MOV(9999,@fb1527d5@.UTIL.LastWrite) ,EQU(@8a3d3297@[0],9999) OTU(@fb1527d5@.CONTROL.ColdBoot) ] ,EQU(@fb1527d5@.UTIL.OddScan,0) NEQ(@fb1527d5@.UTIL.LastService,@fb1527d5@.UTIL.LastWrite) MOV(0,@fb1527d5@.UTIL.LastService) ,MOV(0,@fb1527d5@.UTIL.Mutex) XOR(@fb1527d5@.UTIL.OddScan,1,@fb1527d5@.UTIL.OddScan) ,MOV(@fb1527d5@.UTIL.LastWrite,@8a3d3297@[0]) ];
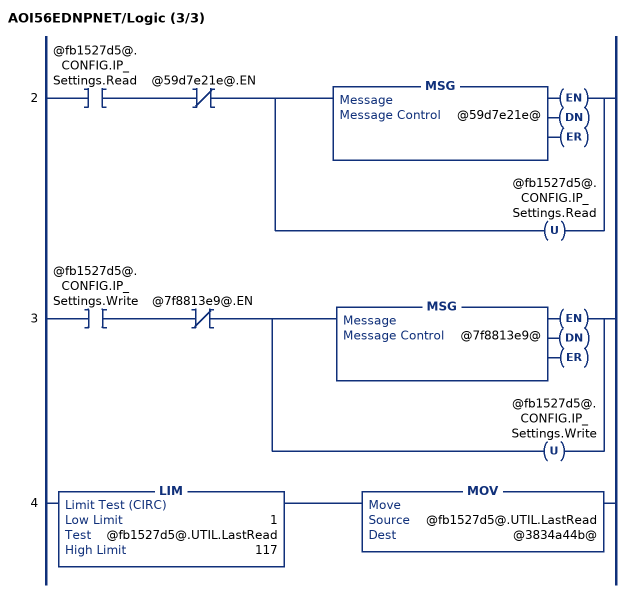
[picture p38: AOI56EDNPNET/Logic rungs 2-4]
   2: XIC(@fb1527d5@.CONFIG.IP_Settings.Read)XIO(@59d7e21e@.EN)[MSG(@59d7e21e@) ,OTU(@fb1527d5@.CONFIG.IP_Settings.Read) ];
   3: XIC(@fb1527d5@.CONFIG.IP_Settings.Write)XIO(@7f8813e9@.EN)[MSG(@7f8813e9@) ,OTU(@fb1527d5@.CONFIG.IP_Settings.Write) ];
   4: LIM(1,@fb1527d5@.UTIL.LastRead,117)MOV(@fb1527d5@.UTIL.LastRead,@3834a44b@);
END_ROUTINE
